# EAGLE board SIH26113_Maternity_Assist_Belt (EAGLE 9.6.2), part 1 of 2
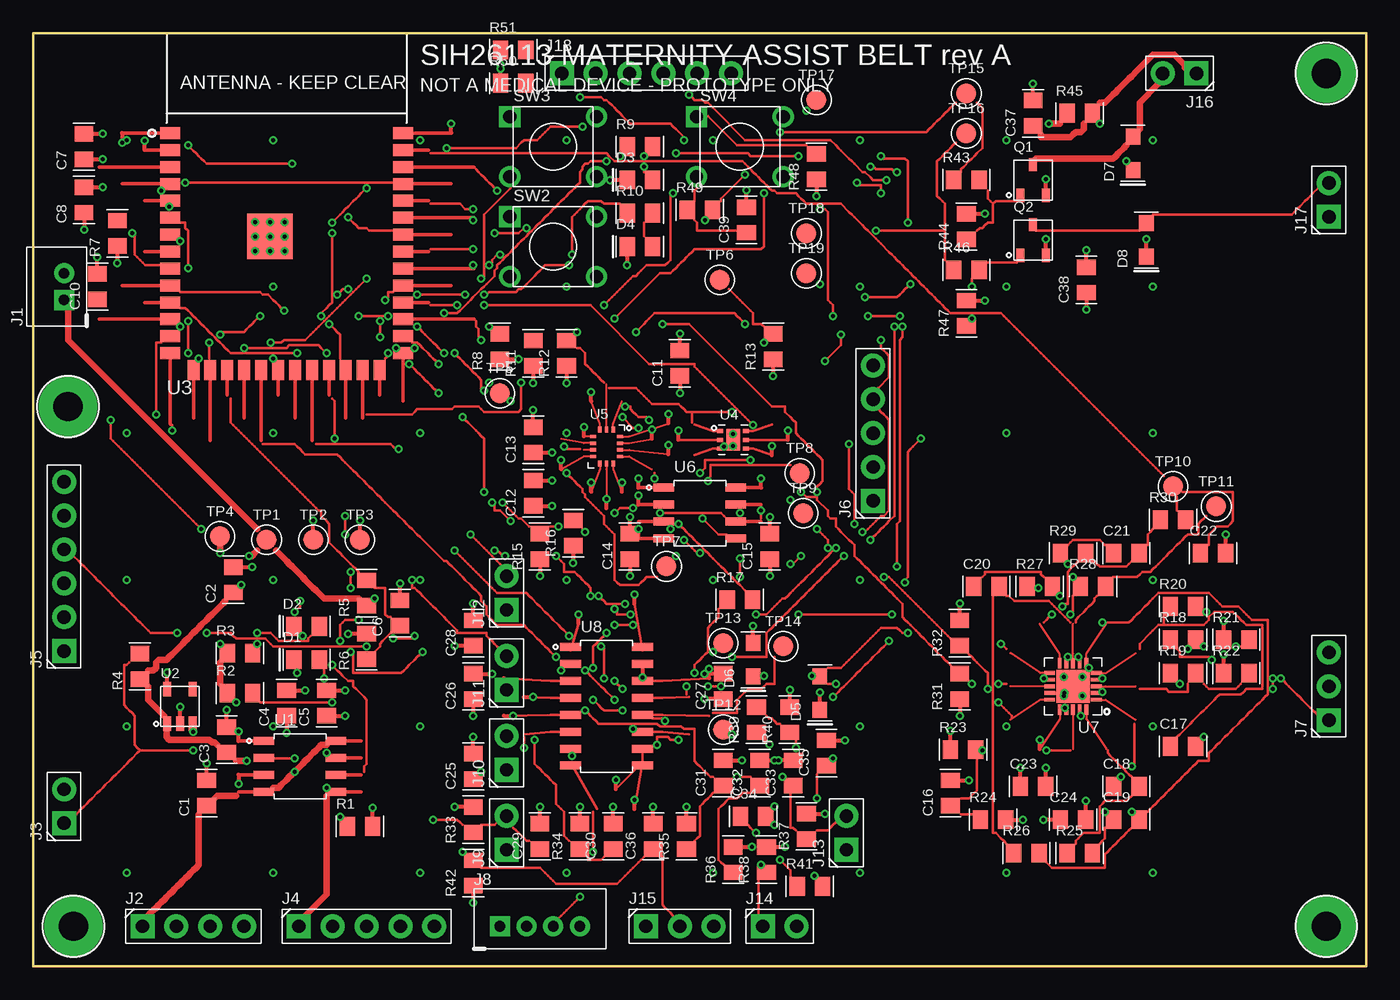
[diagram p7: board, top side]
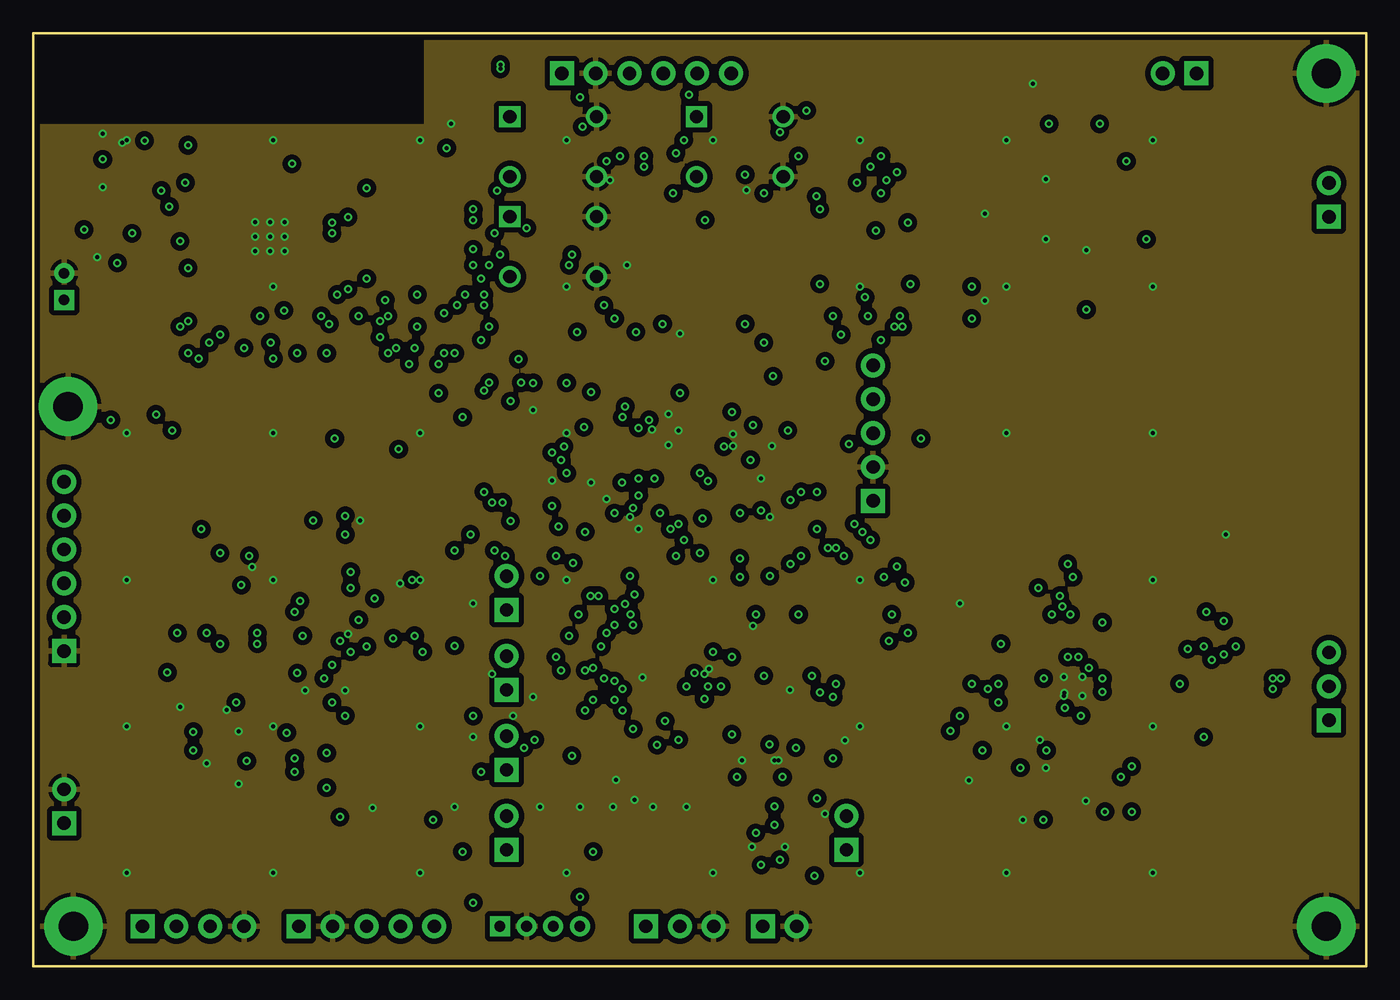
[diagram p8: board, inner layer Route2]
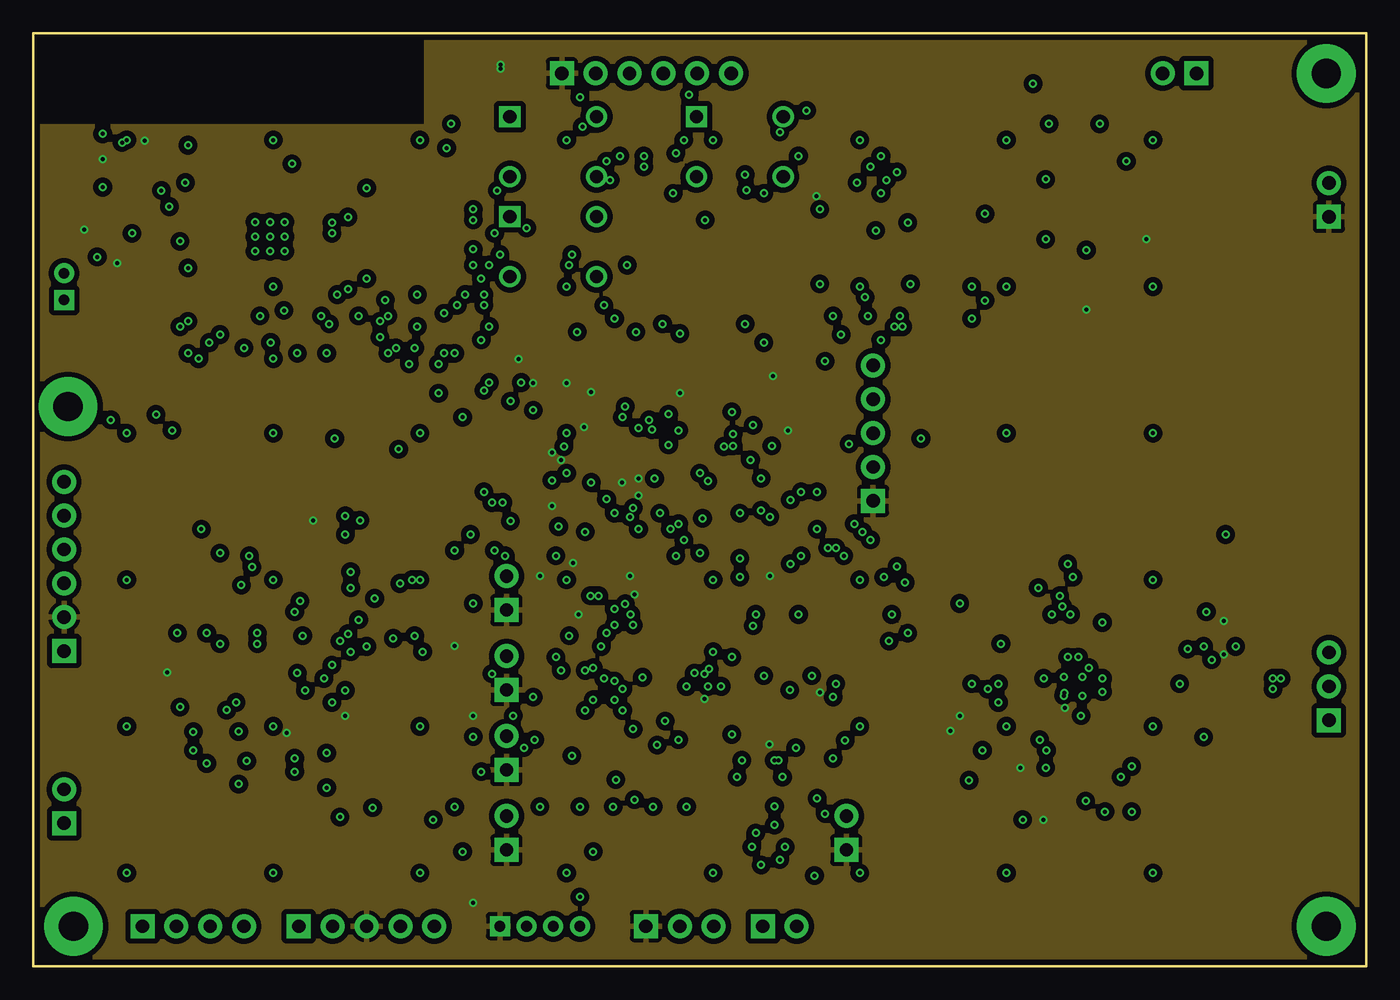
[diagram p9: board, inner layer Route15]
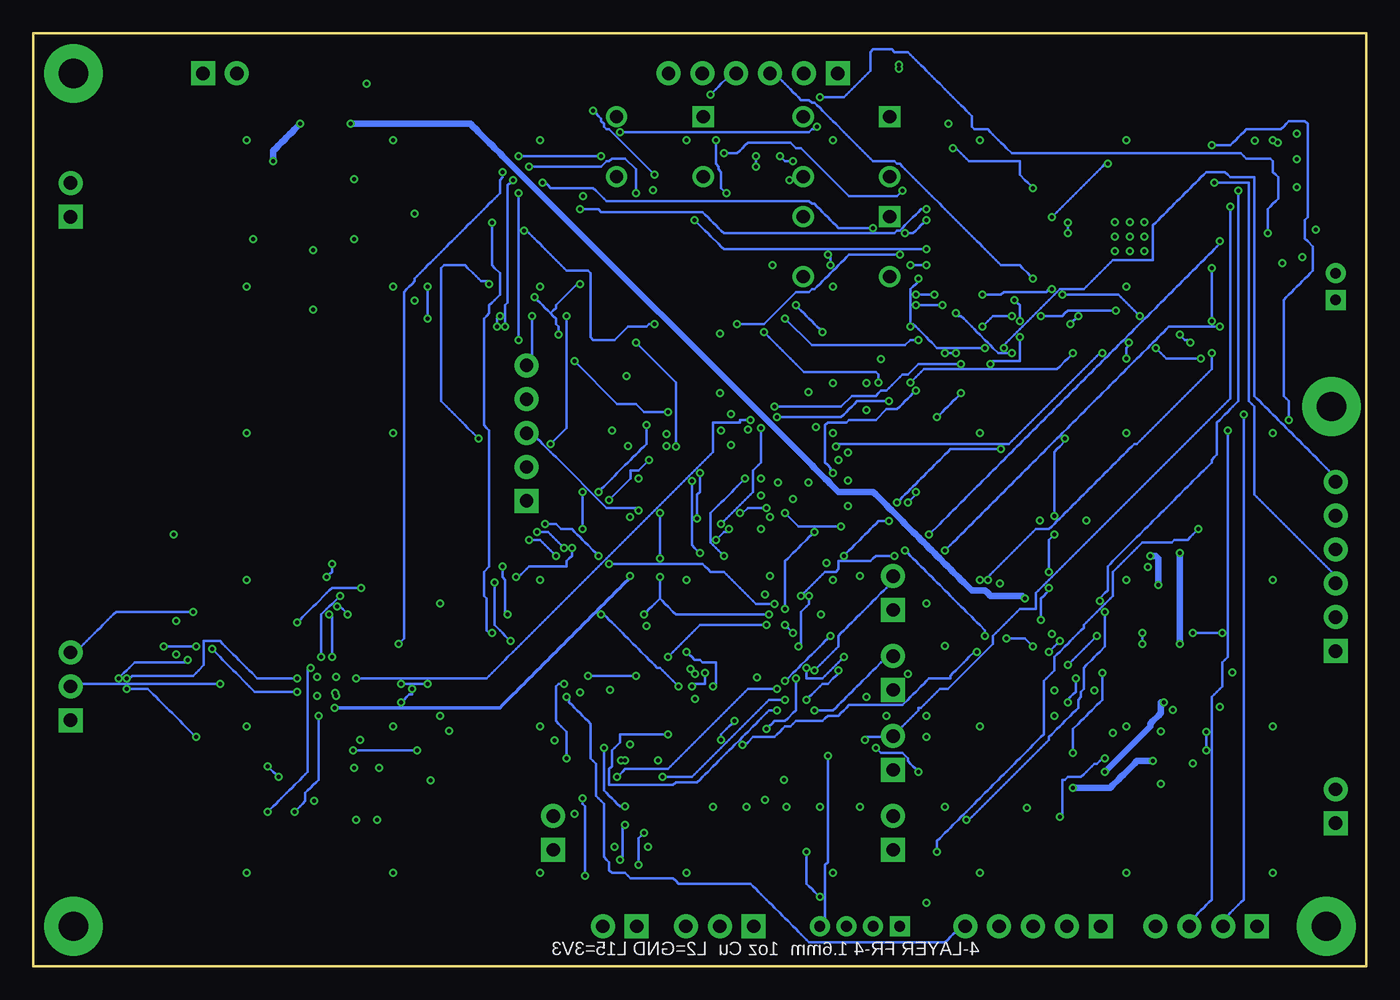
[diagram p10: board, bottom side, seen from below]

Size 100 x 70 mm. Coordinates in mm from the lower left corner, seen from the top.
Outline: 0,0 100,0 100,70 0,70 0,0
Copper layers (1*2*15*16): Top 0.035mm / dielectric 0.36mm / Route2 0.035mm / dielectric 0.71mm / Route15 / Bottom
Design rules "SIH26113_4layer": minimum track width 0.15mm, minimum drill 0.3mm, track to track 0.127mm, track to pad 0.127mm, pad to pad 0.127mm, via to via 0.127mm, smd to smd 0.127mm, copper to edge 0.4mm, drill to drill 0.25mm, minimum pad ring 0.25mm, minimum via ring 0.15mm, thermal gap 0.3mm
Net classes: 0 default: width 0.2 mm, drill 0.3 mm, clearance 0.15 mm; 1 power: width 0.5 mm, drill 0.4 mm, clearance 0.2 mm; 2 motor: width 0.5 mm, drill 0.4 mm, clearance 0.2 mm; 3 analog_ecg: width 0.2 mm, drill 0.3 mm, clearance 0.2 mm
tKeepout: 4 lines
bKeepout: 4 lines
tRestrict: 4 lines
bRestrict: 4 lines
vRestrict: 4 lines

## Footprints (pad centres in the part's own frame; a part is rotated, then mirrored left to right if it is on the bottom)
C0805 = smd 1.15 x 1.4: 1 -0.95,0; 2 0.95,0
LED0805 = smd 1.15 x 1.4: 1 -0.95,0; 2 0.95,0
SOD-123 = smd 1.2 x 1.1: 1 -1.25,0; 2 1.25,0
MOUNT-M2 = drill 2.2 pad 4.4: 1 0,0
JST-PH-2 = drill 0.8 pad 1.5 square: 1 -1,0 | drill 0.8 pad 1.5: 2 1,0
HDR-1X4 = drill 1 pad 1.8 square: 1 -3.81,0 | drill 1 pad 1.8: 2 -1.27,0; 3 1.27,0; 4 3.81,0
HDR-1X2 = drill 1 pad 1.8 square: 1 -1.27,0 | drill 1 pad 1.8: 2 1.27,0
HDR-1X5 = drill 1 pad 1.8 square: 1 -5.08,0 | drill 1 pad 1.8: 2 -2.54,0; 3 0,0; 4 2.54,0; 5 5.08,0
HDR-1X6 = drill 1 pad 1.8 square: 1 -6.35,0 | drill 1 pad 1.8: 2 -3.81,0; 3 -1.27,0; 4 1.27,0; 5 3.81,0; 6 6.35,0
HDR-1X3 = drill 1 pad 1.8 square: 1 -2.54,0 | drill 1 pad 1.8: 2 0,0; 3 2.54,0
JST-PH-4 = drill 0.8 pad 1.5 square: 1 -3,0 | drill 0.8 pad 1.5: 2 -1,0; 3 1,0; 4 3,0
SOT-23-3 = smd 0.6 x 1: 1 -0.95,-1.15; 2 0.95,-1.15; 3 0,1.15
R0805 = smd 1.15 x 1.4: 1 -0.95,0; 2 0.95,0
TACT-6X6-THT = drill 1 pad 1.6 square: 1 -3.25,2.25 | drill 1 pad 1.6: 2 -3.25,-2.25; 3 3.25,2.25; 4 3.25,-2.25
TESTPOINT-1.5 = smd 1.5 x 1.5: TP 0,0
SOIC-8-N = smd 1.55 x 0.6: 1 -2.7,1.905; 2 -2.7,0.635; 3 -2.7,-0.635; 4 -2.7,-1.905; 5 2.7,-1.905; 6 2.7,-0.635; 7 2.7,0.635; 8 2.7,1.905
SOT-23-5 = smd 0.6 x 1.1: 1 -0.95,-1.3; 2 0,-1.3; 3 0.95,-1.3; 4 0.95,1.3; 5 -0.95,1.3
ESP32-S3-WROOM-1 = smd 1.5 x 0.9: 1 -8.75,5.26; 2 -8.75,3.99; 3 -8.75,2.72; 4 -8.75,1.45; 5 -8.75,0.18; 6 -8.75,-1.09; 7 -8.75,-2.36; 8 -8.75,-3.63; 9 -8.75,-4.9; 10 -8.75,-6.17; 11 -8.75,-7.44; 12 -8.75,-8.71; 13 -8.75,-9.98; 14 -8.75,-11.25; 27 8.75,-11.25; 28 8.75,-9.98; 29 8.75,-8.71; 30 8.75,-7.44; 31 8.75,-6.17; 32 8.75,-4.9; 33 8.75,-3.63; 34 8.75,-2.36; 35 8.75,-1.09; 36 8.75,0.18; 37 8.75,1.45; 38 8.75,2.72; 39 8.75,3.99; 40 8.75,5.26 | smd 0.9 x 1.5: 15 -6.985,-12.5; 16 -5.715,-12.5; 17 -4.445,-12.5; 18 -3.175,-12.5; 19 -1.905,-12.5; 20 -0.635,-12.5; 21 0.635,-12.5; 22 1.905,-12.5; 23 3.175,-12.5; 24 4.445,-12.5; 25 5.715,-12.5; 26 6.985,-12.5 | smd 3.4 x 3.4: 41 -1.25,-2.5
WSON-6-DRV0006B = smd 0.45 x 0.3: 1 -0.975,0.65; 2 -0.975,0; 3 -0.975,-0.65; 4 0.975,-0.65; 5 0.975,0; 6 0.975,0.65 | smd 1 x 1.6: 7 0,0
LGA-14L-2.5X3.0 = smd 0.45 x 0.25: 1 1.025,0.75; 2 1.025,0.25; 3 1.025,-0.25; 4 1.025,-0.75; 8 -1.025,-0.75; 9 -1.025,-0.25; 10 -1.025,0.25; 11 -1.025,0.75 | smd 0.25 x 0.45: 5 0.5,-1.275; 6 0,-1.275; 7 -0.5,-1.275; 12 -0.5,1.275; 13 0,1.275; 14 0.5,1.275
LFCSP-20-4X4-P050 = smd 0.8 x 0.28: 1 -1.75,1; 2 -1.75,0.5; 3 -1.75,0; 4 -1.75,-0.5; 5 -1.75,-1; 11 1.75,-1; 12 1.75,-0.5; 13 1.75,0; 14 1.75,0.5; 15 1.75,1 | smd 0.28 x 0.8: 6 -1,-1.75; 7 -0.5,-1.75; 8 0,-1.75; 9 0.5,-1.75; 10 1,-1.75; 16 1,1.75; 17 0.5,1.75; 18 0,1.75; 19 -0.5,1.75; 20 -1,1.75 | smd 2.5 x 2.5: EP 0,0
SOP-16-N = smd 1.55 x 0.6: 1 -2.7,4.445; 2 -2.7,3.175; 3 -2.7,1.905; 4 -2.7,0.635; 5 -2.7,-0.635; 6 -2.7,-1.905; 7 -2.7,-3.175; 8 -2.7,-4.445; 9 2.7,-4.445; 10 2.7,-3.175; 11 2.7,-1.905; 12 2.7,-0.635; 13 2.7,0.635; 14 2.7,1.905; 15 2.7,3.175; 16 2.7,4.445

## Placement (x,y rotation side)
C1  10u  [C0805]  13,13 90 top
C2  10u  [C0805]  15,29 90 top
C3  10u  [C0805]  14.5,17 90 top
C4  10u  [C0805]  19,19.75 90 top
C5  100n  [C0805]  22,19.75 90 top
C6  100n  [C0805]  27.5,26.5 90 top
C7  100n  [C0805]  3.8,61.5 90 top
C8  22u  [C0805]  3.8,57.5 90 top
C10  1u  [C0805]  4.8,51 90 top
C11  100n  [C0805]  48.5,45.25 90 top
C12  100n  [C0805]  37.5,35.5 90 top
C13  100n  [C0805]  37.5,39.5 90 top
C14  100n  [C0805]  44.75,31.5 90 top
C15  1u  [C0805]  55.25,31.5 90 top
C16  100n  [C0805]  68.8,13 90 top
C17  1n  [C0805]  86.25,16.5 0 top
C18  220n  [C0805]  82,13.5 0 top
C19  220n  [C0805]  82,11 0 top
C20  8n2  [C0805]  71.5,28.5 0 top
C21  3n9  [C0805]  82,31 0 top
C22  10n  [C0805]  88.5,31 0 top
C23  100n  [C0805]  75,13.5 0 top
C24  1u  [C0805]  78,11 0 top
C25  100n  [C0805]  33,15 90 top
C26  100n  [C0805]  33,21 90 top
C27  100n  [C0805]  51.75,21 90 top
C28  10u  [C0805]  33,25 90 top
C29  10n  [C0805]  38,9.75 90 top
C30  10n  [C0805]  43.5,9.75 90 top
C31  10n  [C0805]  51.75,14.5 90 top
C32  10n  [C0805]  54.5,14.5 90 top
C33  10n  [C0805]  57,14.5 90 top
C34  100n/50V  [C0805]  54,11.25 0 top
C35  10n  [C0805]  59.5,16 90 top
C36  100n  [C0805]  46.5,9.75 90 top
C37  10u  [C0805]  75,64 90 top
C38  10u  [C0805]  79,51.5 90 top
C39  100n  [C0805]  53.5,56 90 top
D1  RED  [LED0805]  20.5,23 0 top
D2  GRN  [LED0805]  20.5,25.5 0 top
D3  GRN  [LED0805]  45.5,59 0 top
D4  RED  [LED0805]  45.5,54 0 top
D5  1N5819HW  [SOD-123]  59,20.5 90 top
D6  1N5819HW  [SOD-123]  54,23 90 top
D7  1N5819HW  [SOD-123]  82.5,61 90 top
D8  1N5819HW  [SOD-123]  83.5,54.5 90 top
H1  M2  [MOUNT-M2]  3,3 0 top
H2  M2  [MOUNT-M2]  97,3 0 top
H3  M2  [MOUNT-M2]  2.6,42 0 top
H4  M2  [MOUNT-M2]  97,67 0 top
J1  LI-PO 3.7V  [JST-PH-2]  2.3,51 90 top
J2  USB / 5V IN  [HDR-1X4]  12,3 0 top
J3  OFF SW  [HDR-1X2]  2.3,12 90 top
J4  FUEL GAUGE  [HDR-1X5]  25,3 0 top
J5  UART PROG  [HDR-1X6]  2.3,30 90 top
J6  AS5600 SIDE-B  [HDR-1X5]  63,40 90 top
J7  ECG ELECTRODES  [HDR-1X3]  97.2,21 90 top
J8  LOAD CELL  [JST-PH-4]  38,3 0 top
J9  FSR1  [HDR-1X2]  35.5,10 90 top
J10  FSR2  [HDR-1X2]  35.5,16 90 top
J11  FSR3  [HDR-1X2]  35.5,22 90 top
J12  FSR4  [HDR-1X2]  35.5,28 90 top
J13  STRETCH  [HDR-1X2]  61,10 90 top
J14  PIEZO  [HDR-1X2]  56,3 0 top
J15  HALL / LIMIT  [HDR-1X3]  48.5,3 0 top
J16  VIB MOTOR  [HDR-1X2]  86,67 180 top
J17  BUZZER  [HDR-1X2]  97.2,57.5 90 top
J18  MICROSD SPI  [HDR-1X6]  46,67 0 top
Q1  AO3400A  [SOT-23-3]  75,59 0 top
Q2  AO3400A  [SOT-23-3]  75,54.5 0 top
R1  2k4  [R0805]  24.5,10.5 0 top
R2  1k  [R0805]  15.5,20.5 0 top
R3  1k  [R0805]  15.5,23.5 0 top
R4  100k  [R0805]  8,22.5 90 top
R5  470k  [R0805]  25,28 90 top
R6  470k  [R0805]  25,24 90 top
R7  10k  [R0805]  6.3,55 90 top
R8  10k  [R0805]  35,46.5 90 top
R9  1k  [R0805]  45.5,61.5 0 top
R10  1k  [R0805]  45.5,56.5 0 top
R11  4k7  [R0805]  37.5,46 90 top
R12  4k7  [R0805]  40,46 90 top
R13  10k  [R0805]  55.5,46.5 90 top
R15  4k7  [R0805]  38,31.5 90 top
R16  4k7  [R0805]  40.5,32.5 90 top
R17  0R DNP  [R0805]  53,27.5 0 top
R18  330k  [R0805]  86.25,24.5 0 top
R19  330k  [R0805]  86.25,22 0 top
R20  330k  [R0805]  86.25,27 0 top
R21  10M  [R0805]  90.25,24.5 0 top
R22  10M  [R0805]  90.25,22 0 top
R23  10M  [R0805]  69.75,16.25 0 top
R24  10M  [R0805]  72,11 0 top
R25  10M  [R0805]  78.5,8.5 0 top
R26  1M  [R0805]  74.5,8.5 0 top
R27  470k  [R0805]  75.5,28.5 0 top
R28  100k  [R0805]  79.5,28.5 0 top
R29  1M  [R0805]  78,31 0 top
R30  1k  [R0805]  85.5,33.5 0 top
R31  100k  [R0805]  69.5,21 90 top
R32  100k  [R0805]  69.5,25 90 top
R33  10k  [R0805]  33,11 90 top
R34  10k  [R0805]  41,9.75 90 top
R35  10k  [R0805]  49,9.75 90 top
R36  10k  [R0805]  52.5,8 90 top
R37  10k  [R0805]  58,10.5 90 top
R38  10M  [R0805]  55,8 90 top
R39  1M  [R0805]  54.25,18.5 90 top
R40  1M  [R0805]  56.75,18.5 90 top
R41  100k  [R0805]  58.25,6 0 top
R42  10k  [R0805]  33,7 90 top
R43  100R  [R0805]  70,59 0 top
R44  100k  [R0805]  70,55.5 90 top
R45  0R  [R0805]  78.5,64 0 top
R46  100R  [R0805]  70,52.25 0 top
R47  100k  [R0805]  70,49 90 top
R48  10k  [R0805]  58.75,60 90 top
R49  1k  [R0805]  50,56.75 0 top
R50  10k  [R0805]  36,66.25 0 top
R51  10k  [R0805]  36,68.75 0 top
SW2  RESET  [TACT-6X6-THT]  39,54 0 top
SW3  BOOT  [TACT-6X6-THT]  39,61.5 0 top
SW4  SOS  [TACT-6X6-THT]  53,61.5 0 top
TP1  VBAT  [TESTPOINT-1.5]  17.5,32 0 top
TP2  3V3  [TESTPOINT-1.5]  21,32 0 top
TP3  GND  [TESTPOINT-1.5]  24.5,32 0 top
TP4  VBUS  [TESTPOINT-1.5]  14,32.25 0 top
TP5  IO3  [TESTPOINT-1.5]  35,43 0 top
TP6  TMP_ALERT  [TESTPOINT-1.5]  51.5,51.5 0 top
TP7  IMU_INT1  [TESTPOINT-1.5]  47.5,30 0 top
TP8  AS_OUT  [TESTPOINT-1.5]  57.5,37 0 top
TP9  AS_PGO  [TESTPOINT-1.5]  57.75,34 0 top
TP10  ECG_OUT  [TESTPOINT-1.5]  85.5,36 0 top
TP11  ECG_REF  [TESTPOINT-1.5]  88.75,34.5 0 top
TP12  HX_BASE  [TESTPOINT-1.5]  51.75,17.75 0 top
TP13  HX_XO  [TESTPOINT-1.5]  51.75,24.25 0 top
TP14  HX_DOUT  [TESTPOINT-1.5]  56.25,24 0 top
TP15  MOTOR_EN  [TESTPOINT-1.5]  70,65.5 0 top
TP16  BUZZER_EN  [TESTPOINT-1.5]  70,62.5 0 top
TP17  SOS_GPIO  [TESTPOINT-1.5]  58.75,65 0 top
TP18  I2C_SDA  [TESTPOINT-1.5]  58,55 0 top
TP19  I2C_SCL  [TESTPOINT-1.5]  58,52 0 top
U1  TP4056  [SOIC-8-N]  20,15 0 top
U2  AP2112K-3.3  [SOT-23-5]  11,19.5 0 top
U3  ESP32-S3-WROOM-1-N8R2  [ESP32-S3-WROOM-1]  19,57.25 0 top
U4  TMP117  [WSON-6-DRV0006B]  52.5,39.5 0 top
U5  LSM6DSOX  [LGA-14L-2.5X3.0]  43,39 0 top
U6  AS5600  [SOIC-8-N]  50,34 0 top
U7  AD8232  [LFCSP-20-4X4-P050]  78,21 180 top
U8  HX711  [SOP-16-N]  43,19.5 0 top

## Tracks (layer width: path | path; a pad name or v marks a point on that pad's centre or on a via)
3V3  (via drill 0.3 pad 0.55, 0.3 pad 0.6)
  Top 0.15: U5.5 43.5,37.3 44.15,35.6 | U5.8 41.3,38.25 39.6,37.27 | U5.11 41.3,39.75 | U5.12 42.5,40.7 41.85,42.4
  Top 0.2: U4.5 54,39.5 56.6,39.5 | U8.1 40.3,23.7 40.9,25.7 | U8.16 45.7,23.7 45.1,27.2 | U8.3 38.8,21.41 35.3,21.6
  Top 0.25: U3.2 8.35,61.24 | U6.1 45.4,35.91 | U6.2 45.4,34.63
  Top 0.3: U2.5 v10.05,22.05 | C4.1 v19,17.52 | C5.1 v23.4,18.8 | TP2.TP v21,33.45 | 8.35,61.24 v8.35,61.94 | C7.1 v5.2,60.55 | C8.1 v3.8,55.27 | R7.1 v6.3,52.77 | R8.1 v36.4,45.55 | R11.1 v37.5,43.77 | R12.1 v40,43.77 | 56.6,39.5 v56.6,40.2 | C11.1 v48.5,43.02 | R13.1 v55.5,44.27 | 44.15,35.6 v44.15,36.3 | 39.6,37.27 v39.6,37.98 | 41.3,39.75 v41.3,40.45 | 41.85,42.4 v41.85,43.1 | C12.1 v38.9,34.55 | C13.1 v38.9,38.55 | R15.1 v38,29.27 | R16.1 v40.5,30.27 | 45.4,35.91 v45.4,36.6 | 45.4,34.63 v45.4,35.34 | C14.1 v44.75,29.27 | C15.1 v55.25,29.27 | R21.1 v89.3,25.9 | R22.1 v89.3,23.4 | R23.1 v68.8,17.65 | R31.1 v69.5,18.77 | C23.1 v74.05,14.9 | C24.1 v75.78,11 | 40.9,25.7 v40.9,26.4 | 35.3,21.6 v35.3,20.9 | 45.1,27.2 v45.1,27.9 | C26.1 v33,18.77 | C27.1 v50.35,20.05 | C28.1 v31.6,24.05 | R39.1 v55.24,16.64 | D5.1 v59,20.55 | R42.1 v33,4.78 | D8.1 v83.5,54.55 | C38.1 v79,49.27 | R48.1 v58.75,57.77 | R50.1 v35.05,67.65 | R51.1 v35.05,67.35
  Bottom 0.25: v77.4,19.4 65,19.4 64.8,19.6 64.6,19.8 64.4,20 64.2,20.2 64,20.4 63.8,20.6 63.6,20.8 63.4,21 63.2,21.2 63,21.4 62.8,21.6 62.6,21.8 62.4,22 62.2,22.2 62,22.4 61.8,22.6 61.6,22.8 61.4,23 61.2,23.2 61,23.4 60.8,23.6 60.6,23.8 60.4,24 60.2,24.2 60,24.4 59.8,24.6 59.6,24.8 59.4,25 59.2,25.2 59,25.4 58.8,25.6 58.6,25.8 58.4,26 58.2,26.2 58,26.4 57.8,26.6 57.6,26.8 57.4,27 57.2,27.2 57,27.4 56.8,27.6 56.6,27.8 56.4,28 56.2,28.2 56,28.4 55.8,28.6 55.6,28.8 55.4,29
  pour Route15 (isolate 0.4): 0.5,0.5 99.5,0.5 99.5,69.5 29.5,69.5 29.5,63 0.5,63
ANG2_OUT  (via drill 0.3 pad 0.6)
  Top 0.2: 51.4,26.8 51.4,26.2 51.2,26 51,25.8 50.8,25.6 50.6,25.4 50.6,23.6 50.4,23.4 50.2,23.2 50,23 49.8,22.8 49.6,22.6 v49.6,22 | v50.6,21 v51.6,21 | v57.4,26.4 v64.4,26.4 | v64.8,30 64.8,33.2 65,33.4 65,47 65.2,47.2 v65.2,48 | v65,48.8 v62.6,48.8
  Bottom 0.2: v49.6,22 49.6,21.2 50.4,21.2 v50.6,21 | v51.6,21 51.8,21.2 52,21.4 52.4,21.8 52.6,22 52.8,22.2 53,22.4 53.2,22.4 53.4,22.6 53.6,22.8 53.8,23 54,23.2 54.4,23.6 54.6,23.8 54.8,24 55,24.2 55.4,24.6 55.6,24.8 55.8,25 56,25.2 56.4,25.6 56.6,25.8 56.8,26 57,26.2 57.2,26.4 v57.4,26.4 | v64.4,26.4 64.6,26.6 64.6,29 64.8,29.2 v64.8,30 | v65.2,48 65.2,48.6 v65,48.8 | v62.6,48.8 62.6,45.8
ANG_SCL  (via drill 0.3 pad 0.6)
  Top 0.2: 53,34.4 v53,34 | v53,30.6 v53,29.2 | v54.2,26.4 55,26.4 55.4,26.8 55.6,27 55.8,27.2 56,27.4 56.2,27.6 56.4,27.6 56.6,27.8 56.8,28 57,28.2 57.4,28.6 57.6,28.8 57.8,29 58,29.2 58.4,29.6 58.6,29.8 58.8,30 59,30.2 59.4,30.6 59.6,30.8 59.8,31 60,31.2 v60.2,31.4 | v62.2,32.6 62.4,32.6 62.6,32.8 62.8,33 63,33.2 63.2,33.4 63.4,33.6 63.6,33.8 63.8,33.8 64.2,34.2 64.2,41 64,41.2 63.8,41.4 63.6,41.6 63.4,41.8 | 41.2,32.8 v41.4,32.6 | v43.6,26.8 43.8,26.6 43.8,26.4 v44.8,26.4 | v34.6,55 36.4,55 36.8,55.4 v37,55.4 | v61.8,58.8 62,58.6 63.6,58.6 v63.6,58 | v63.6,47 63.6,46.4 63.8,46.2 64,46 64.2,45.8 64.2,44.2 63.4,43.4
  Top 0.25: U3.35 33.05,56.16 | U6.7 54.6,34.63
  Bottom 0.2: v53,34 v53,30.6 | v53,29.2 53,27.6 | 53,27.6 53.4,27.2 53.6,27 53.8,26.8 54,26.6 v54.2,26.4 | v60.2,31.4 60.4,31.6 60.6,31.8 60.8,32 61,32.2 61.2,32.4 61.4,32.6 v62.2,32.6 | v41.4,32.6 41.6,32.4 41.8,32.2 42,32 42.4,31.6 42.6,31.4 42.8,31.2 43,31 43.4,30.6 43.6,30.4 v43.6,26.8 | v44.8,26.4 51.8,26.4 52,26.6 52.4,27 52.6,27.2 52.8,27.4 53,27.6 | v33,56 33.2,55.8 33.4,55.6 33.6,55.4 33.8,55.2 34,55 v34.6,55 | v37,55.4 39.6,55.4 39.8,55.6 40,55.8 40.2,56 40.4,56.2 40.6,56.4 40.8,56.6 41,56.8 41.2,57 41.4,57.2 41.6,57.2 41.8,57.4 57,57.4 57.2,57.6 57.8,58.2 58,58.4 61.2,58.4 61.4,58.6 61.6,58.8 v61.8,58.8 | v63.6,58 v63.6,47
ANG_SDA  (via drill 0.3 pad 0.6)
  Top 0.2: 54.6,33.6 v54.6,34.2 | 38.8,33 v39.4,33 | v43.6,34 44,34.4 v45,34.4 | v47,34 51.6,34 51.8,33.8 52,33.6 | 21.2,39.2 26.8,39.2 27,39 27.2,38.8 v27.4,38.8 | v35.2,34.8 35.4,34.6 35.6,34.4 35.8,34.2 36,34 36.2,33.8 36.4,33.6 36.6,33.6 37.2,33
  Top 0.25: U3.22 20.91,39.45 | U6.6 54.6,33.37
  Bottom 0.2: v54.6,34.2 54.6,34.4 57,34.4 60.8,38.2 61,38.4 61.2,38.6 61.8,39.2 62,39.4 62.2,39.6 | v39.4,33 42.6,33 v43.6,34 | v45,34.4 46.4,34.4 46.8,34 v47,34 | v27.4,38.8 31.2,38.8 31.4,38.6 31.6,38.4 32,38 32.2,37.8 32.4,37.6 32.6,37.4 32.8,37.2 33,37 33.2,36.8 33.4,36.6 33.6,36.4 33.8,36.2 34,36 34.2,35.8 34.4,35.6 34.6,35.4 34.8,35.2 35,35 v35.2,34.8
AS_OUT  (via drill 0.3 pad 0.6)
  Top 0.2: 47.8,33 v47.8,32.8 | v48.8,32 49,31.8 49.4,31.4 49.6,31.2 49.8,31 v50,31 | v50.6,36.4 50.6,36.6 50.8,36.8 50.8,37.6 56.8,37.6
  Top 0.25: U6.3 45.4,33.37
  Bottom 0.2: v47.8,32.8 47.8,32.6 48.2,32.6 v48.8,32 | v50,31 50.2,31.2 50.4,31.4 50.6,31.6 v50.6,36.4
AS_PGO  (via drill 0.3 pad 0.6)
  Top 0.2: 52,32.4 51.4,32.4 v50.2,33.6 | v50,37 50.2,37.2 50.4,37.4 50.4,38 v53.8,38 | v56.8,35 57,34.8
  Bottom 0.2: v50.2,33.6 50.2,35.4 50,35.6 v50,37 | v53.8,38 54.6,37.2 55.2,37.2 55.2,36.6 v56.8,35
BUZZ_G  (via drill 0.3 pad 0.6)
  Top 0.2: 70.4,51.6 v70.4,51 | 73.8,52.8 71.6,52.8
  Bottom 0.2: v70.4,51 v70.4,48.6
BUZZ_N
  Top 0.2: 84,56.4 94.4,56.4 94.6,56.6 94.8,56.8 95,57 95.4,57.4 95.6,57.6 95.8,57.8 96,58 96.4,58.4 | 75.2,55.2 83,55.2
BUZZER_EN  (via drill 0.3 pad 0.6)
  Top 0.2: 68.4,53 68.4,57.2 68.2,57.4 68,57.6 67.8,57.8 67.8,60.4 68,60.6 68.2,60.8 68.4,61 68.6,61.2 68.8,61.4 69,61.6 69.2,61.8 | 25,41.4 28.4,41.4 28.6,41.6 28.8,41.8 31.4,41.8 31.6,42 33.4,42 33.6,41.8 33.8,41.6 36.4,41.6 36.6,41.8 v36.6,43.8 | v45.2,47.6 45.8,48.2 46,48.4 46.2,48.6 46.6,49 52.6,49 52.8,48.8 53,48.6 53.2,48.4 v53.4,48.2 | v63.2,55.2 68.4,55.2
  Top 0.25: U3.25 24.71,41.15
  Bottom 0.2: v36.6,43.8 36.6,44.4 36.8,44.6 42.2,44.6 42.8,45.2 43,45.4 43.2,45.6 43.8,46.2 44,46.4 44.2,46.6 44.8,47.2 45,47.4 v45.2,47.6 | v53.4,48.2 53.8,48.2 54,48 55.4,48 56.4,47 58,47 58.2,47.2 58.2,52 58.4,52.2 60,52.2 60.2,52.4 60.4,52.6 60.6,52.8 60.8,53 61,53.2 61.2,53.4 61.4,53.6 61.6,53.8 61.8,54 62,54.2 62.2,54.4 62.4,54.6 62.6,54.8 62.8,55 63,55.2 v63.2,55.2
CHG_PROG  (via drill 0.3 pad 0.6)
  Top 0.2: 18,15.6 v19.6,15.6
  Bottom 0.2: v19.6,15.6 19.8,15.6 20,15.4 20.2,15.2 20.4,15.2 20.6,15 21,14.6 21.2,14.4 21.4,14.2 22.4,14.2 22.6,14 22.8,14 22.8,11.4 v23,11.2
ECG_FR  (via drill 0.3 pad 0.6)
  Top 0.15: U7.15 75.55,20 73.3,18.5
  Top 0.2: 73.4,18.6 73.4,18.8 73.2,19 73,19.2 72.8,19.4 72.6,19.6 v72.4,19.8 | v71.6,20.8 71.6,22 71.4,22.2 70.8,22.8 70.6,23 70.4,23.2 70.2,23.4 | v34.2,52.6 34.4,52.8 34.4,53 34.8,53.4 v35,53.4 | v47.2,48.2 49.2,48.2 55.4,42 56.4,42 56.4,41.6 56.8,41.2 57,41 57.2,40.8 57.2,40 57.4,39.8 57.6,39.6 57.8,39.4 58,39.2 58.2,39 58.4,38.8 58.6,38.6 58.8,38.4 59,38.2 59.2,38 59.2,36.4 59,36.2 58.8,36 v58.8,35.6 | v58.8,32.8 59,32.6 59.2,32.4 59.4,32.2 59.6,32 v59.6,31.4 | v63.8,29.2 64.2,29.2 64.4,29 64.6,28.8 64.8,28.6 65.2,28.2 65.4,28 65.6,27.8 65.8,27.6 66.2,27.2 66.4,27 66.6,26.8 66.8,26.6 67.2,26.2 67.4,26 67.6,25.8 67.8,25.6 68.2,25.2 68.4,25 68.6,24.8 68.8,24.6
  Top 0.25: U3.32 33.05,52.35
  Bottom 0.2: v72.4,19.8 72.2,20 72,20.2 71.8,20.4 71.6,20.4 v71.6,20.8 | v33,52.6 v34.2,52.6 | v35,53.4 38.8,53.4 39,53.2 39.2,53 39.4,52.8 39.6,52.6 39.8,52.4 40,52.2 40.2,52 40.4,51.8 40.6,51.6 40.8,51.4 41,51.2 41.2,51 41.4,50.8 41.6,50.8 41.8,50.6 42.8,50.6 45.2,48.2 v47.2,48.2 | v58.8,35.6 v58.8,32.8 | v59.6,31.4 59.6,30.8 59.8,30.6 60,30.4 60,30 62.8,30 63,29.8 63.4,29.4 63.6,29.2 v63.8,29.2
ECG_HPDRIVE  (via drill 0.3 pad 0.6)
  Top 0.15: U7.1 80.45,20 82.7,18.5
  Top 0.2: 82.6,18.2 82.6,15.2 v82.4,15
  Bottom 0.2: v82.4,15 82,14.6 81.8,14.4 v81.6,14.2
ECG_HPSENSE
  Top 0.15: U7.20 79,18.55 80.5,16.3
  Top 0.2: 80.6,16.2 80.6,16 80.8,15.8 81,15.6 81.2,15.4 81.4,15.2 81.6,15 81.8,14.8 82,14.6 82.2,14.4 82.4,14.2 | 78.2,9.2 78.2,9.4 78.4,9.6 78.8,10 80,10 80,12 80.2,12.2 80.4,12.4 82,12.4 82.2,12.6 82.4,12.8
ECG_IAOUT  (via drill 0.3 pad 0.6)
  Top 0.2: 80.4,9.6 80.4,10.4 80.4,9.6 | 80.4,9.6 80.2,9.4 | 80.2,9.4 80,9.2 80.2,9.4 | 80.4,9.6 80.2,9.4
  Bottom 0.2: v78.6,18.8 78.6,14 78.8,13.8 79,13.6 79.2,13.4 79.4,13.2 79.6,13 79.6,12.4 79.8,12.2 80,12 v80.4,11.6
ECG_LA  (via drill 0.3 pad 0.6)
  Top 0.2: 85.8,23.8 86,23.6 86,23.2 88.2,23.2 v88.4,23 | v93.6,21.6 93.8,21.4 94,21.2 94.2,21 94.8,20.4 95,20.2 95.2,20 95.8,19.4 96,19.2 96.2,19 96.4,18.8
  Bottom 0.2: v88.4,23 88.6,22.8 92.4,22.8 92.8,22.4 93,22.2 93.2,22 v93.6,21.6
ECG_LA_F  (via drill 0.3 pad 0.6)
  Top 0.2: 90.6,24 v90.2,24
  Bottom 0.2: v90.2,24 v87.8,24 | v80.2,20.6 83.4,20.6 83.8,21 84,21.2 84.8,22 85,22.2 85.8,23 86,23.2 v86.6,23.8
ECG_LOD_N  (via drill 0.3 pad 0.6)
  Top 0.15: U7.11 75.55,22 73.3,23.5
  Top 0.2: 73,23.8 72.8,24 v72.6,24.2 | v64.8,59.6 64.6,59.6 64.4,59.8 63.2,59.8 63,60 v62.8,60 | v54.8,58 54.8,54 54.6,53.8 49.6,53.8 49.4,53.6 49.2,53.4 49,53.2 48.8,53 48.6,52.8 48.4,52.6 48.2,52.4 48,52.2 47.8,52 47,52 v43.6,48.6 | v33.6,47 33.4,47.2 33.4,47.8 33.2,48 33.2,48.4
  Top 0.25: U3.29 33.05,48.54
  Bottom 0.2: v72.6,24.2 72.2,24.6 72.2,50.6 72,50.8 71.8,51 71.6,51.2 71.4,51.4 71.4,51.6 71.2,51.8 71,52 70.8,52.2 70.6,52.4 70.4,52.6 70.2,52.8 70,53 69.8,53.2 69.6,53.4 69.4,53.6 69.2,53.8 69,54 68.8,54.2 68.6,54.4 68.4,54.6 68.2,54.8 68,55 67.8,55.2 67.6,55.4 67.4,55.6 67.2,55.8 67,56 66.8,56.2 66.6,56.4 66.4,56.6 66.2,56.8 66,57 65.8,57.2 65.6,57.4 65.4,57.6 65.2,57.8 65,58 65,59 64.8,59.2 v64.8,59.6 | v62.8,60 57.4,60 57,60.4 56.8,60.4 56.6,60.6 55.6,60.6 54.8,59.8 v54.8,58 | v43.6,48.6 41.6,46.6 34.6,46.6 34.2,47 v33.6,47
ECG_LOD_P  (via drill 0.3 pad 0.6)
  Top 0.2: v46.2,41 46,41.2 45.4,41.2 45.2,41.4 45,41.6 44.8,41.8 44.8,42 v44.4,42 | v30.4,45.2 30.2,45.4 30,45.6 29.8,45.8 29.6,46 29.2,46.4 29,46.6 28.8,46.8 28.4,46.8
  Bottom 0.2: v75.8,21.6 66,21.6 65.8,21.8 65.6,22 65.4,22.2 64.8,22.8 64.6,23 64.4,23.2 64,23.6 63.8,23.8 63.6,24 63.4,24.2 63,24.6 62.8,24.8 62.6,25 62.4,25.2 62,25.6 61.8,25.8 61.6,26 61.4,26.2 61,26.6 60.8,26.8 60.6,27 60.4,27.2 60,27.6 59.8,27.8 59.6,28 59.4,28.2 59,28.6 58.8,28.8 58.6,29 58.4,29.2 58,29.6 57.8,29.8 57.6,30 57.4,30.2 57,30.6 56.8,30.8 56.6,31 56.4,31.2 56,31.6 55.8,31.8 55.6,32 55.4,32.2 55.2,32.4 55,32.6 54.8,32.8 54.6,33 54.4,33.2 54.2,33.4 54,33.6 53.8,33.8 53.6,34 53.4,34.2 53.2,34.4 53,34.6 52.8,34.8 52.6,35 52.4,35.2 52.2,35.4 52,35.6 51.8,35.8 51.6,36 51.4,36.2 51.2,36.4 51,36.6 50.8,36.8 50.6,37 50.4,37.2 50.2,37.4 50,37.6 49.8,37.8 49.6,38 49.4,38.2 49.2,38.4 49,38.6 49,40.8 47,40.8 47,41 v46.2,41 | v44.4,42 39.4,42 38.6,42.8 36.8,42.8 36.6,43 36.4,43.2 36,43.2 35.8,43.4 35.6,43.6 35,44.2 34.8,44.4 34.4,44.4 33.6,45.2 v30.4,45.2
ECG_OPM  (via drill 0.3 pad 0.6)
  Top 0.2: 77.6,30.4 v77.6,30.2 | 80.4,31.6 80,32 78,32 77.8,31.8 77.6,31.6 | v77.8,26.4 78,26.4 78,27.8
  Bottom 0.2: v77.6,30.2 77.6,29.6 77.8,29.4 v78,29.2 | v77.6,23.2 77.6,26.2 v77.8,26.4
ECG_OPP  (via drill 0.3 pad 0.6)
  Top 0.2: 71.4,29.4 71.2,29.2 71.4,29.4 | 71.4,29.4 71.4,29.6 | 71.4,29.6 75.6,29.6 | 75.6,29.6 75.6,29.4 | 75.6,29.4 75.8,29.2 75.6,29.4 | 71.4,29.4 71.4,29.6 | 71.4,29.6 75.6,29.6 | 75.6,29.6 75.6,29.4
  Bottom 0.2: v78.4,23.2 78.4,26.4 78,26.8 77.8,27 77.6,27.2 v77,27.8
ECG_OUT
  Top 0.2: 85.8,34.2 85.8,35.2 | 88.2,31.6 88.2,32.4 88.6,32.8 88.8,33 89.6,33 89.8,33.2 90,33.4 90,35.6 86.2,35.6 | 29.8,61 43,61 43.2,60.8 43.6,60.4 53.2,60.4 53.4,60.2 53.6,60 53.8,59.8 54,59.6 54.2,59.4 54.4,59.2 54.6,59 54.8,58.8 55,58.6 55.2,58.4 55.4,58.2 55.6,58.2 55.8,58 57.2,58 57.4,57.8 57.6,57.6 57.8,57.4 58,57.2 60.6,57.2 61.2,56.6 61.4,56.4 61.6,56.2 62.2,55.6 62.4,55.4 62.6,55.2 63.2,54.6 63.4,54.4 63.6,54.2 64.2,53.6 64.4,53.4 64.6,53.2 64.8,53 65,52.8 65.2,52.6 65.4,52.4 65.6,52.2 65.8,52 66,51.8 66.2,51.6 66.4,51.4 66.6,51.2 66.8,51 67,50.8 67.2,50.6 67.4,50.4 67.6,50.2 67.8,50 68,49.8 68.2,49.6 68.4,49.4 68.6,49.2 68.8,49 72.6,49 72.8,48.8 73,48.6 73.2,48.4 73.6,48 73.8,47.8 74,47.6 74.2,47.4 74.6,47 74.8,46.8 75,46.6 75.2,46.4 75.6,46 75.8,45.8 76,45.6 76.2,45.4 76.6,45 76.8,44.8 77,44.6 77.2,44.4 77.6,44 77.8,43.8 78,43.6 78.2,43.4 78.6,43 78.8,42.8 79,42.6 79.2,42.4 79.6,42 79.8,41.8 80,41.6 80.2,41.4 80.6,41 80.8,40.8 81,40.6 81.2,40.4 81.6,40 81.8,39.8 82,39.6 82.2,39.4 82.6,39 82.8,38.8 83,38.6 83.2,38.4 83.6,38 83.8,37.8 84,37.6 84.2,37.4 84.4,37.2 84.6,37 84.8,36.8
  Top 0.25: U3.39 29.65,61.24
ECG_OUT_RAW  (via drill 0.3 pad 0.6)
  Top 0.15: U7.10 77,23.45 75.5,25.7
  Top 0.2: 83.6,32.4 83.6,31.6 83.6,32.4 | 83.6,32.4 83.8,32.6 | 83.8,32.6 84,32.8 83.8,32.6 | 79.8,30.2 79.6,30.4 79.8,30.2 | 79.8,30.2 80,30 | 80,30 82,30 | 82,30 82.2,30.2 | 82.2,30.2 82.4,30.4 82.2,30.2 | 83.6,32.4 83.8,32.6 | 79.8,30.2 80,30 | 80,30 82,30 | 82,30 82.2,30.2 | 75.8,25.8 76,26 76.2,26.2 v76.4,26.4 | v77.2,27 77.4,27.2 77.6,27.2 77.6,29.6 77.8,29.8 78,30 78.2,30.2 78.4,30.4
  Bottom 0.2: v76.4,26.4 76.8,26.8 77,27 v77.2,27
ECG_RA  (via drill 0.3 pad 0.6)
  Top 0.2: 85.8,21.2 v86,21.2
  Bottom 0.2: v86,21.2 96.4,21.2
ECG_RA_F
  Top 0.15: U7.3 80.45,21 82.7,21
  Top 0.2: 90.6,21.2 90.4,21 90.2,20.8 88.2,20.8 88,21 87.8,21.2 | 83,20.8 85,20.8 85.2,20.6 86.6,20.6 86.6,21.2
ECG_REFIN  (via drill 0.3 pad 0.6)
  Top 0.15: U7.18 78,18.55 78,16.3
  Top 0.2: 70.8,13.2 70.8,15.6 70.8,13.2 | 70.8,13.2 70.6,13 | 70.6,13 70.2,12.6 | 70.2,12.6 69.6,12.6 70.2,12.6 | 70.8,13.2 70.6,13 | 70.6,13 70.2,12.6 | 77.8,16.2 v76,16.2 | 70.4,11.4 69.6,11.4 70.4,11.4
  Bottom 0.2: v76,16.2 v71.2,16.2
ECG_REFOUT
  Top 0.15: U7.8 78,23.45 78,25.7
  Top 0.2: 81,29.2 82.8,29.2 83,29.4 83.2,29.6 83.8,29.6 84,29.8 84.2,30 84.4,30.2 84.8,30.6 85,30.8 85.2,31 85.4,31.2 85.8,31.6 86,31.8 86.2,32 86.4,32.2 86.6,32.4 87.4,32.4 87.4,33.2 87.6,33.4 87.8,33.6 88,33.8 | 78.2,25.8 78.2,26 78.4,26.2 78.8,26.6 79,26.8 79.2,27 79.4,27.2 79.6,27.4 79.6,27.6 79.8,27.8 | 73,27.8 73.2,27.8 73.6,27.4 76.2,27.4 76.4,27.2 76.6,27 76.8,26.8 77,26.6 77.4,26.2 77.6,26 77.8,25.8 | 73,9.2 72.8,9.4 72.6,9.6 72.2,10 72,10 72,27.8
ECG_RL  (via drill 0.3 pad 0.6)
  Top 0.2: 87.8,26.6 v88,26.6
  Bottom 0.2: v88,26.6 93.8,26.6 94,26.4 94.2,26.2 94.4,26 94.8,25.6 95,25.4 95.2,25.2 95.4,25 95.8,24.6 96,24.4 96.2,24.2 96.4,24
ECG_RLD
  Top 0.15: U7.5 80.45,22 82.7,23.5
  Top 0.2: 83,23.8 83,24.2 83.8,25 84,25.2 84.4,25.6 87.8,25.6 88,25.8 88.2,26 88.2,26.2 88.6,26.6 90,26.6 90.4,26.2 90.6,26 90.8,25.8 91,25.6 92.2,25.6 92.2,20.8 91,20.8 90.8,20.6 90.6,20.4 89,20.4 88.8,20.2 88.6,20 88,19.4 87.8,19.2 87.6,19 87,18.4 86.8,18.2 86,17.4 85.8,17.2 | 84.8,26.4 84.8,25.6
ECG_RLDFB  (via drill 0.3 pad 0.6)
  Top 0.2: v93,21.6 v93,20.8
  Bottom 0.2: v80.2,21.6 83.2,21.6 83.6,22 83.8,22.2 84,22.4 84.6,23 84.8,23.2 85,23.4 85.6,24 85.8,24.2 86,24.4 87.2,24.4 87.2,22.6 87.6,22.2 87.8,22 88,21.8 92.6,21.8 92.8,21.6 v93,21.6 | v93,20.8 91.4,20.8 91,20.4 90.8,20.2 90.6,20 90,19.4 89.8,19.2 89.6,19 89,18.4 88.8,18.2 88,17.4 v87.8,17.2
ECG_SDN  (via drill 0.3 pad 0.6)
  Top 0.15: U7.13 75.55,21 73.3,21
  Top 0.2: 73,21.2 v72.4,21.2 | v70.4,21.2 70.2,21.4 | 29.8,49.6 v31.8,49.6 | v33.8,49.6 41.8,49.6 46.2,45.2 49.6,45.2 49.6,45 49.8,44.8 50,44.6 50.2,44.4 50.4,44.2 50.6,44 50.8,43.8 51,43.6 51.2,43.4 51.4,43.2 51.6,43 51.8,42.8 52,42.6 52.2,42.4 52.4,42.2 52.6,42 52.8,41.8 53,41.6 53.2,41.4 53.4,41.2 53.6,41 53.8,40.8 v54,40.6 | v57.6,35.6 58,35.2 58.8,35.2 58.8,35 59.6,34.2 59.6,33.8 59.8,33.6 60.2,33.6 60.2,33 60.4,32.8 60.6,32.6 61.2,32 61.4,31.8 61.6,31.6 61.6,30.8 61.8,30.6 62,30.4 62.2,30.2 62.4,30 62.6,29.8 62.8,29.6 63,29.4 63.2,29.2 63.4,29 63.6,28.8 63.8,28.6 64,28.4 64.2,28.2 64.4,28 64.6,27.8 64.8,27.6 65.2,27.2 65.2,26.2 65.4,26 65.6,25.8 65.8,25.6 66.2,25.2 66.4,25 66.6,24.8 66.8,24.6 67.2,24.2 67.4,24 67.6,23.8 67.8,23.6 68.2,23.2 68.4,23 68.6,22.8 68.8,22.6
  Top 0.25: U3.30 29.65,49.81
  Bottom 0.2: v72.4,21.2 v70.4,21.2 | v31.8,49.6 v33.8,49.6 | v54,40.6 54,39.2 54.2,39 54.4,38.8 54.6,38.6 54.8,38.4 55,38.2 55.2,38 55.4,37.8 55.6,37.6 56.2,37 56.4,36.8 56.6,36.6 57.2,36 57.4,35.8 v57.6,35.6
ECG_SW  (via drill 0.3 pad 0.6)
  Top 0.15: U7.6 79,23.45 80.5,25.7
  Top 0.2: 82.2,10.2 82.4,10.4 82.2,10.2 | 82.2,10.2 82,10 | 82,10 81.8,9.8 | 81.8,9.8 81.6,9.6 | 81.6,9.6 81.4,9.4 | 81.4,9.4 81.2,9.2 | 81.2,9.2 81,9 | 81,9 80.8,8.8 | 80.8,8.8 80.6,8.6 | 80.6,8.6 80.4,8.4 | 80.4,8.4 80.4,7.4 | 80.4,7.4 76.4,7.4 | 76.4,7.4 76,7.8 76.4,7.4 | 80.6,25.8 82.2,25.8 82.4,26 82.6,26.2 82.8,26.4 83,26.6 83.4,27 83.6,27.2 83.8,27.4 84,27.6 84.4,28 88.2,28 88.8,27.4 89,27.2 89.2,27 90.4,27 90.8,26.6 91,26.4 91.2,26.2 91.4,26 92.6,26 92.6,20.4 92.4,20.2 92.2,20 92,19.8 91.8,19.6 91.4,19.2 91.2,19 91,18.8 90.8,18.6 90.6,18.4 90.4,18.2 90,17.8 89.8,17.6 89.6,17.4 89.4,17.2 89,16.8 88.8,16.6 88.6,16.4 88.4,16.2 88.2,16 88.2,15.4 87.4,15.4 87.2,15.2 87,15 86.8,14.8 86.6,14.6 86.4,14.4 86.2,14.2 86,14 85.8,13.8 85.6,13.6 85.4,13.4 85.2,13.2 85,13 84.8,12.8 84.6,12.6 84.4,12.4 84.2,12.2 84,12 83.8,11.8 83.6,11.6 | 82.2,10.2 82,10 | 82,10 81.8,9.8 | 81.8,9.8 81.6,9.6 | 81.6,9.6 81.4,9.4 | 81.4,9.4 81.2,9.2 | 81.2,9.2 81,9 | 81,9 80.8,8.8 | 80.8,8.8 80.6,8.6 | 80.6,8.6 80.4,8.4 | 80.4,8.4 80.4,7.4 | 80.4,7.4 76.4,7.4 | 75.2,28.4 v75.4,28.4
  Bottom 0.2: v79.2,22.4 79.4,22.4 79.4,14.6 79.6,14.4 79.8,14.2 80,14 80.4,13.6 80.6,13.4 80.8,13.2 81,13 81.4,12.6 81.6,12.4 81.8,12.2 82,12 v82.4,11.6 | v75.4,28.4 77.6,28.4 77.8,28.2 78,28 78.8,27.2 79,27 79.8,26.2 80,26 v80.2,25.8
ESP_EN
  Top 0.25: U3.3 4.95,59.97
ESP_IO0  (via drill 0.3 pad 0.6)
  Top 0.2: v33.6,51.6 33.8,51.6 33.8,56.4 35.8,58.4 | 28.4,46.4 v28.6,46.4
  Top 0.25: U3.27 27.75,42.4
  Bottom 0.2: v34.2,48 34.2,50.8 34,51 33.8,51.2 33.6,51.4 v33.6,51.6 | v28.6,46.4 32.2,46.4 32.6,46.8 32.8,47 33,47.2 33.6,47.8 33.8,48 34,48.2 34.2,48.2 | 2.8,37.2 3,37.4 3.4,37.8 3.6,38 3.8,38.2 4,38.4 4.2,38.6 4.4,38.8 4.6,39 4.8,39.2 5,39.4 5.2,39.6 5.4,39.8 5.6,40 5.8,40.2 6,40.4 6.2,40.6 6.4,40.8 6.6,41 6.8,41.2 7,41.4 7.2,41.6 7.4,41.8 7.6,42 7.8,42.2 8,42.4 8.2,42.6 8.4,42.8 8.4,59.2 10.2,59.2 10.4,59.4 10.6,59.6 12,59.6 12.2,59.4 12.4,59.2 12.6,59 12.8,58.8 13,58.6 13.2,58.4 13.4,58.2 13.6,58 13.8,57.8 14,57.6 14.2,57.4 14.4,57.2 14.6,57 14.8,56.8 15,56.6 15.2,56.4 15.4,56.2 15.6,56 15.8,55.8 16,55.6 16,53 19,53 19.2,52.8 19.4,52.6 19.6,52.4 20,52 20.2,51.8 20.4,51.6 20.6,51.4 21,51 21.2,50.8 23,50.8 23.2,50.6 23.4,50.4 23.8,50 24,49.8 24.2,49.6 24.4,49.4 24.8,49 25,48.8 25.2,48.6 25.4,48.4 25.8,48 26,47.8 26.2,47.6 26.4,47.4 26.8,47 27,46.8 27.2,46.6 v27.2,46.4
FSR1_ADC  (via drill 0.3 pad 0.6)
  Top 0.2: 33.6,10.6 34.6,10.6 34.8,10.8 | 37.2,9.4 37,9.4 36.8,9.6 36.4,10 36.2,10.2 36,10.4 | v20,27.4 20,27 v19.6,26.6 | v30,11 31.8,11 32,10.8 32.2,10.6
  Top 0.25: U3.4 6.65,58.7
  Bottom 0.2: v9.6,58.2 9.6,42.4 10,42 10.2,41.8 10.4,41.6 10.6,41.4 11,41 11.2,40.8 11.2,38.4 11.4,38.2 11.6,38 11.6,37.8 12,37.4 12.2,37.2 12.4,37 12.6,36.8 13,36.4 13.2,36.2 13.4,36 13.6,35.8 14,35.4 14.2,35.2 14.4,35 14.6,34.8 15,34.4 15.2,34.2 15.4,34 15.6,33.8 16,33.4 16.2,33.2 16.4,33 16.6,32.8 17,32.4 17.2,32.2 19,30.4 19.2,30.2 19.4,30 19.4,28.2 19.6,28 20,27.6 v20,27.4 | v19.6,26.6 19.6,24 20,23.6 20.2,23.4 20.4,23.2 20.6,23 21,22.6 21.2,22.4 21.2,20.8 21.4,20.6 21.4,20.2 21.6,20 21.6,19.4 21.8,19.2 22,19 22.2,18.8 22.6,18.4 22.8,18.2 23,18 23.2,17.8 23.6,17.4 23.8,17.2 23.8,17 24,16.8 24.2,16.6 24.4,16.4 24.6,16.2 25,15.8 25.2,15.6 25.4,15.4 25.6,15.2 25.8,15 26,14.8 26.2,14.6 26.4,14.4 26.6,14.2 26.8,14 27,13.8 27.2,13.6 27.4,13.4 27.6,13.2 27.8,13 28,12.8 28.2,12.6 28.4,12.4 28.6,12.2 28.8,12 29,11.8 29.2,11.6 29.4,11.4 29.6,11.2 29.8,11 v30,11
FSR2_ADC  (via drill 0.3 pad 0.6)
  Top 0.2: 40.2,9.4 40,9.6 39.8,9.8 39.8,11.6 39.6,11.8 39.4,12 39.2,12.2 39.2,13.6 39,13.8 38.8,14 38.6,14.2 38.4,14.4 38.2,14.6 38,14.8 37.8,15 37.6,15.2 v37.6,17 | 42.8,8.2 42.6,8 41.6,8 41.6,8.2
  Top 0.25: U3.5 8.35,57.43
  Bottom 0.2: v37.6,17 37.6,17.2 36.4,17.2 | v10.2,57 10.2,42.6 10.4,42.4 10.6,42.2 10.8,42 11,41.8 11.2,41.6 11.4,41.4 11.6,41.2 11.8,41 12,40.8 12.2,40.6 12.4,40.4 12.6,40.2 12.8,40 13,39.8 13.2,39.6 13.4,39.4 13.6,39.2 13.8,39 14,38.8 14.2,38.6 14.4,38.4 14.6,38.2 14.8,38 15,37.8 15.2,37.6 15.4,37.4 15.6,37.2 15.8,37 16,36.8 16.2,36.6 16.4,36.4 16.6,36.2 16.8,36 17,35.8 17.2,35.6 17.4,35.4 17.6,35.2 17.8,35 18,34.8 18.2,34.6 18.4,34.4 18.6,34.2 18.8,34 19,33.8 19.2,33.6 19.4,33.4 19.6,33.2 19.8,33 20,32.8 20.2,32.6 20.4,32.4 20.6,32.2 20.8,32 21,31.8 21.2,31.6 21.6,31.2 21.8,31 22,30.8 22.2,30.6 22.6,30.2 22.8,30 23,29.8 23.2,29.6 23.6,29.2 23.8,29 24,28.8 24.2,28.6 24.6,28.2 24.8,28 24.8,26.8 26,26.8 26.2,26.6 26.6,26.2 26.8,26 27,25.8 27.2,25.6 27.6,25.2 27.8,25 28,24.8 28,24.2 31.4,20.8 32,20.8 32.2,20.6 32.4,20.4 32.6,20.2 32.8,20 33,19.8 33.2,19.6 33.4,19.4 33.6,19.4 33.6,19.2 33.8,19 34,18.8 34.2,18.6 34.4,18.4 34.6,18.2 34.8,18 35,17.8
FSR3_ADC  (via drill 0.3 pad 0.6)
  Top 0.2: 51,14.2 50.8,14.2 50.6,14.4 50.4,14.6 50,15 49.8,15.2 49.6,15.4 49.6,17.8 48.8,17.8 48.6,18 47,18 46.8,18.2 42.4,18.2 42.2,18.4 42,18.6 41.8,18.8 41.6,19 v41.4,19.2 | 49.6,9.4 49.8,9.6 50,9.8 50,12 50.2,12.2 50.4,12.4 50.6,12.6 50.8,12.8 51,13 | 11,55.8 11.4,55.8 11.4,55.4 11.6,55.2 v11.6,52.4 | v11.6,48.4 v11.6,46 | v28.4,29 28.4,28.4 28.6,28.4 28.8,28.2 29,28 29.2,27.8 29.8,27.2 30,27 30.2,26.8 30.8,26.2 31,26 31.2,25.8 31.8,25.2 31.8,25 34,25 34,24.8 34.2,24.6 34.4,24.4 34.6,24.2 34.8,24 35,23.8
  Bottom 0.2: v41.4,19.2 40,19.2 39.8,19.4 39.6,19.6 39.4,19.8 39.2,20 39,20.2 38.8,20.4 38.6,20.6 38.4,20.8 38.2,21 38,21.2 37.8,21.4 37.4,21.8 37.2,22 37,22.2 36.8,22.4 36.4,22.8 | v11.6,52.4 v11.6,48.4 | v11.6,46 11.6,44.8 11.8,44.6 12,44.4 12.2,44.2 12.4,44 12.6,43.8 12.8,43.6 13,43.4 13.2,43.2 13.4,43 13.6,42.8 13.8,42.6 14,42.4 14.2,42.2 14.4,42 14.6,41.8 14.8,41.6 15,41.4 15.2,41.2 15.4,41 15.6,40.8 15.8,40.6 16,40.4 16.2,40.2 16.4,40 16.6,39.8 16.8,39.6 17,39.4 17.2,39.2 17.4,39.2 17.6,39 17.8,38.8 18,38.6 18.2,38.4 18.4,38.2 18.6,38 18.8,37.8 19,37.6 19.2,37.4 19.4,37.2 19.6,37 19.8,36.8 20,36.6 20.2,36.4 20.4,36.2 20.6,36 20.8,35.8 21,35.6 21.2,35.4 21.4,35.2 21.6,35 21.8,34.8 22,34.6 22.2,34.4 22.4,34.2 22.6,34 22.8,33.8 23,33.6 23.2,33.4 23.4,33.2 23.6,33 23.8,32.8 24.8,32.8 25,32.6 25.2,32.4 25.4,32.2 25.6,32 26,31.6 26.2,31.4 26.4,31.2 26.6,31 27,30.6 27.2,30.4 27.4,30.2 27.6,30 28,29.6 28.2,29.4 28.4,29.2 v28.4,29
FSR4_ADC  (via drill 0.3 pad 0.6)
  Top 0.2: 53.8,14.2 v52.8,14.2 | v43.6,20 43.4,20.2 43,20.6 42.8,20.8 42.6,21 42.4,21.2 42,21.6 41.8,21.8 41.6,22 v41.4,22.2 | 51.8,7.6 51.6,7.8 51.4,8 51.4,11.8 51.6,12 51.8,12.2 52,12.4 52.2,12.6 52.8,12.6 53,12.8 53.2,13 53.8,13 | v32.8,32.4 33.2,32 33.4,31.8 33.8,31.4 34,31.2 34.2,31 34.4,30.8 34.8,30.4 35,30.2 35.2,30
  Bottom 0.2: v52.8,14.2 50.6,14.2 50.4,14.4 50.2,14.6 50,14.8 49.8,15 49.6,15.2 49.4,15.4 49.2,15.6 49,15.8 48.8,16 48.6,16.2 48.4,16.4 48,16.8 47.8,17 47.6,17.2 47.4,17.4 47,17.8 46.8,18 46.6,18.2 46.4,18.4 46,18.8 45.8,19 45.6,19.2 45.4,19.4 45,19.8 44.8,20 v43.6,20 | v41.4,22.2 41,22.6 40.8,22.8 40.6,23 40.4,23.2 40,23.6 39.8,23.8 39.6,24 39.6,24.8 39.4,25 39.2,25.2 39,25.4 38.8,25.6 38.6,25.8 38.4,26 38.2,26.2 38,26.4 37.8,26.6 37.4,27 37.2,27.2 37,27.4 36.8,27.6 36.4,28 36.2,28.2 36,28.4 | v11,54.4 11,54.2 11.2,54 11.4,53.8 11.6,53.6 11.8,53.4 12,53.2 12.2,53 12.4,52.8 12.6,52.6 12.8,52.4 13,52.2 13.2,52 13.4,51.8 13.6,51.6 13.8,51.4 14,51.2 14.2,51 14.4,50.8 14.6,50.6 14.8,50.4 15,50.2 15.2,50 15.4,49.8 15.6,49.6 15.8,49.4 16.2,49 16.4,48.8 16.6,48.6 16.8,48.4 17.2,48 17.4,47.8 17.6,47.6 17.8,47.4 18.2,47 18.4,46.8 18.6,46.6 18.8,46.4 19,46.2 19.2,46 19.4,45.8 19.6,45.6 19.8,45.4 20,45.2 20.2,45 20.4,44.8 20.6,44.6 20.8,44.4 21,44.2 21.2,44 21.4,43.8 21.6,43.6 21.8,43.4 22,43.2 22.2,43 22.4,42.8 22.6,42.6 22.8,42.4 23,42.2 23.2,42 23.4,41.8 23.6,41.6 23.8,41.4 24,41.2 24.2,41 24.4,40.8 24.6,40.6 24.8,40.4 25,40.2 25.2,40 25.4,39.8 25.6,39.6 25.8,39.4 26,39.2 26.2,39 26.4,38.8 26.6,38.6 26.8,38.4 27,38.2 27.2,38 27.4,37.8 27.8,37.4 28,37.2 28.2,37 28.4,36.8 28.8,36.4 29,36.2 29.2,36 29.4,35.8 29.8,35.4 30,35.2 30.2,35 30.4,34.8 30.8,34.4 31,34.2 31.2,34 31.4,33.8 31.8,33.4 32,33.2 v32.8,32.4
GND  (via drill 0.3 pad 0.55, 0.3 pad 0.6)
  Top 0.15: U5.3 44.7,38.75 47.65,38.42 | U5.2 44.7,39.25 46.4,39.58 | U5.1 44.7,39.75 47.65,40.73 | U5.7 42.5,37.3 41.85,35.6 | U5.6 43,37.3 43,34.35 | U7.16 77,18.55 75.5,16.3
  Top 0.2: U4.2 51,39.5 48.4,39.5 | U4.4 54,38.85 55.4,38.35 | U8.5 38.8,18.86 35.3,18.8 | U8.4 38.8,20.14 36.8,20.2 | U8.10 45.7,15.3 | 45.7,15.3 43.7,13.3 | U8.9 45.7,15.3 | 45.7,15.3 45.1,11.8 | U8.14 47.2,21.41 50.7,21.6
  Top 0.25: U1.1 15.4,16.91 | U1.3 15.4,14.37 | U3.1 6.65,62.51 | U3.40 31.35,62.51 | U6.4 45.4,32.09 | U6.8 54.6,35.91
  Top 0.3: 15.4,16.91 v15.4,17.61 | 15.4,14.37 v15.4,13.66 | R1.2 v25.45,11.9 | C1.2 v13,15.22 | C2.2 v16.4,29.95 | U2.2 v11,19.45 | C3.2 v14.5,19.23 | C4.2 v20.4,20.7 | C5.2 v23.4,20.7 | R6.2 v23.6,24.95 | C6.2 v27.5,28.73 | TP3.TP v24.5,33.45 | 6.65,62.51 v6.65,61.81 | 31.35,62.51 v31.35,63.21 | C7.2 v5.2,62.45 | C8.2 v5.2,58.45 | C10.2 v4.8,53.23 | D3.1 v43.27,59 | D4.1 v44.55,52.6 | 48.4,39.5 v48.4,40.2 | 55.4,38.35 v55.4,39.05 | C11.2 v48.5,47.48 | 47.65,40.73 v47.65,41.42 | 46.4,39.58 v46.4,40.27 | 47.65,38.42 v47.65,39.12 | 43,34.35 v43,35.05 | 41.85,35.6 v41.85,36.3 | C12.2 v38.9,36.45 | C13.2 v37.5,41.73 | 45.4,32.09 v45.4,32.8 | 54.6,35.91 v54.6,36.6 | C14.2 v44.75,33.73 | C15.2 v55.25,33.73 | U7.14 v77.35,20.5 | 75.5,16.3 v75.5,17 | R24.2 v74.22,11 | C16.2 v70.2,13.95 | C22.2 v89.45,32.4 | R32.2 v69.5,27.23 | C23.2 v75.95,14.9 | C24.2 v78.95,12.4 | 36.8,20.2 v37.5,20.2 | 35.3,18.8 v36,18.8 | 45.1,11.8 v45.1,12.5 | 43.7,13.3 v43.7,14 | 50.7,21.6 v50.7,22.3 | U8.15 v45.7,21.68 | C25.2 v33,17.23 | C26.2 v34.4,21.95 | C27.2 v50.35,21.95 | C28.2 v33,27.23 | R33.2 v31.6,11.95 | C29.2 v38,11.97 | R34.2 v41,11.97 | C30.2 v43.5,11.97 | R35.2 v49,11.97 | C31.2 v53.15,15.45 | R36.2 v53.9,8.95 | C32.2 v55.9,15.45 | R37.2 v59.4,11.45 | C33.2 v55.6,15.45 | R38.2 v56.4,8.95 | R40.2 v56.75,20.73 | C35.2 v60.9,16.95 | D6.2 v54,25.55 | C36.2 v46.5,11.97 | Q1.2 v75.95,59.05 | R44.2 v71.4,56.45 | C37.2 v75,66.22 | Q2.2 v75.95,54.55 | R47.2 v71.4,49.95 | C38.2 v79,53.73 | C39.2 v53.5,58.23
  other vias: 16.65,53.65 16.65,54.75 16.65,55.85 17.75,53.65 17.75,54.75 17.75,55.85 18.85,53.65 18.85,54.75 18.85,55.85 52.5,39.95 52.5,39.05 78.7,21.7 77.3,21.7 78.7,20.3 77.3,20.3 7,7 7,18 7,29 7,40 7,62 18,7 18,18 18,29 18,40 18,51 18,62 29,7 29,18 29,29 29,40 29,62 40,7 40,29 40,40 40,51 40,62 51,7 51,29 51,62 62,7 62,18 62,29 62,51 62,62 73,7 73,18 73,40 73,51 73,62 84,7 84,18 84,29 84,40 84,51 84,62
  pour Route2 (isolate 0.4): 0.5,0.5 99.5,0.5 99.5,69.5 29.5,69.5 29.5,63 0.5,63
HALL_LIMIT  (via drill 0.3 pad 0.6)
  Top 0.2: 47.2,8.2 47.2,4.6 47.4,4.4 47.6,4.2 47.8,4 48,3.8 | 33.6,7.4 38,7.4 38.4,7 38.6,6.8 38.8,6.6 39,6.4 39.2,6.2 43.8,6.2 44,6.4 44.4,6.8 44.6,7 44.8,7.2 45,7.4 45.4,7.8 45.6,8 45.8,8.2 | 27,55.2 25.2,55.2 25,55.4 24.4,55.4 24.2,55.6 24,55.8 23.8,56 v23.6,56.2 | v19.4,60.2 13,60.2 12.8,60.4 12.6,60.6 12.4,60.8 12.2,61 12,61.2 11.8,61.4 v11.6,61.6 | v5.8,41 5.8,39.6 6,39.4 6.4,39 6.6,38.8 6.8,38.6 7,38.4 7.4,38 7.6,37.8 7.8,37.6 8,37.4 8.2,37.2 8.4,37 8.6,36.8 8.8,36.6 9,36.4 9.2,36.2 9.4,36 9.6,35.8 10,35.4 10.2,35.2 10.4,35 10.6,34.8 11,34.4 11.2,34.2 11.4,34 11.6,33.8 12,33.4 12.2,33.2 12.4,33 v12.6,32.8
  Top 0.25: U3.34 31.35,54.89
  Bottom 0.2: v23.6,56.2 23.4,56.4 23.2,56.6 23,56.8 22.8,57 22.4,57.4 22.2,57.6 22,57.8 21.8,58 21.4,58.4 21.2,58.6 21,58.8 20.8,59 20.4,59.4 20.2,59.6 20,59.8 19.8,60 19.6,60.2 v19.4,60.2 | v11.6,61.6 10.2,61.6 10,61.8 9.8,62 9.6,62.2 9.4,62.4 9.2,62.6 9,62.8 6.4,62.8 6.2,63 6,63.2 5.8,63.4 4.6,63.4 4.4,63.2 4.4,56.2 4.6,56 4.6,54.6 4.4,54.4 4,54 4,52.2 4.2,52 4.4,51.8 4.6,51.6 4.8,51.4 5,51.2 5.2,51 5.4,50.8 5.6,50.6 5.8,50.4 6,50.2 6.2,50 6.2,42.8 6,42.6 5.8,42.4 v5.8,41 | v12.6,32.8 13,32.4 13.2,32.2 13.4,32 14.4,32 14.6,31.8 16.8,31.8 17.2,31.4 17.4,31.2 17.6,31 18.2,30.4 18.4,30.2 18.6,30 19,29.6 19,27.8 19.2,27.6 19.6,27.2 19.8,27 20,26.8 20.2,26.6 20.6,26.2 20.8,26 21,25.8 21.2,25.6 21.2,25.4 21.4,25.2 21.6,25 22,24.6 22.2,24.4 22.4,24.2 22.6,24 23,23.6 23.2,23.4 23.4,23.2 23.4,22.2 23.6,22 24,21.6 24.2,21.4 24.2,17.4 24.4,17.2 25,16.6 25.2,16.4 25.4,16.2 26,15.6 26.2,15.4 26.4,15.2 26.6,15 27,14.6 27.2,14.4 27.4,14.2 27.6,14 28,13.6 28.2,13.4 28.4,13.2 28.6,13 29,12.6 29.2,12.4 29.4,12.2 29.6,12 30,11.6 30.2,11.4 30.4,11.2 30.6,11 31,10.6 31.2,10.4 31.4,10.2 31.6,10 32,9.6 32.2,9.4 v32.2,8.6
HX_BASE  (via drill 0.3 pad 0.6)
  Top 0.2: 39.6,22.4 v39.6,22.2 | v42,20 42.4,19.6 42.6,19.4 42.8,19.2 v44.2,19.2
  Bottom 0.2: v39.6,22.2 39.6,22 39.8,21.8 40,21.6 40.4,21.2 40.8,21.2 41,21 41.4,20.6 41.6,20.4 41.8,20.2 v42,20 | v44.2,19.2 44.8,19.2 45,19 45.4,18.6 45.6,18.4 45.8,18.2 46,18 46.4,17.6 46.6,17.4 46.8,17.2 47,17 47.4,16.6 47.6,16.4 47.8,16.2 48,16 48.4,15.6 48.6,15.4 48.8,15.2 49,15 49.4,14.6 49.6,14.4 49.8,14.2 50,14 50.2,13.8 51.8,13.8 52,13.6 56.8,13.6 56.8,14.8 56.6,15 56.6,16.2 56.4,16.4 56,16.8 56,17.4 v52.4,17.4
HX_DOUT  (via drill 0.3 pad 0.6)
  Top 0.2: U8.12 47.2,18.86 50.7,18.8 | 51,19 52.8,19 52.8,20 53,20.2 53.4,20.6 53.6,20.8 54.6,20.8 54.8,21 55,21.2 55.6,21.2 55.6,23.2 | 22.4,42.6 22.6,42.4 v22.6,39.6 | v23.4,33.8 v23.4,32.4 | v23.8,29.6 v23.8,28.4 | v24.4,26 23.4,26 23.2,25.8 23,25.6 v23,24.4 | v23.8,23.6 24,23.4 24,22 27.6,22 27.8,22.2 28,22.4 28.2,22.6 28.6,23 28.8,23.2 29,23.4 v29.2,23.6 | v46.8,16.6 46.8,17.2 47.6,17.2 47.8,17 v48.4,17 | v47.4,18.4 47.2,18.6 46.4,18.6
  Top 0.25: U3.23 22.18,42.85
  Bottom 0.2: v22.6,39.6 22.6,39.4 23,39 23.2,38.8 23.4,38.6 v23.4,33.8 | v23.4,32.4 23.6,32.2 23.8,32 v23.8,29.6 | v23.8,28.4 23.8,28.2 24,28 24.2,27.8 24.4,27.6 v24.4,26 | v23,24.4 23,24.2 23.2,24.2 23.4,24 v23.8,23.6 | v29.2,23.6 29.4,23.6 29.8,23.2 30,23 30.2,22.8 30.8,22.2 31,22 31.2,21.8 31.2,21.6 32.8,21.6 33,21.4 33.2,21.2 33.4,21 33.8,20.6 34,20.4 34.2,20.2 34.4,20 34.8,19.6 38.8,19.6 39,19.4 39.2,19.2 39.4,19 39.6,18.8 40.4,18.8 40.6,18.6 40.8,18.4 42.8,18.4 43,18.2 43.2,18 43.6,18 43.8,17.8 44,17.6 44.2,17.4 44.4,17.2 46,17.2 46.4,16.8 46.6,16.6 v46.8,16.6 | v48.4,17 48.4,17.4 48,17.8 47.8,18 47.6,18.2 v47.4,18.4
HX_SCK  (via drill 0.3 pad 0.6)
  Top 0.2: U8.11 47.2,17.59 49.2,17.4 | v42.8,21.6 42.8,23.8 v42.6,24 | v41.8,27.8 41.8,28.4 41.6,28.6 41.4,28.8 41.2,29 41,29.2 40.8,29.4 40.6,29.6 39.8,29.6 39.8,30.2 39.6,30.4 39.4,30.6 v39.2,30.8 | v35.8,33.4 35,34.2 34.6,34.2 34.6,34.6 v34.4,34.8 | v33.8,35.6 33.8,39.6 33.6,39.8 33.4,40 33.2,40.2 32.6,40.8 32.4,41 v32.2,41.2 | v30.4,43 30.2,43.2 30,43.4 29.8,43.6 29.6,43.8 29.4,44 29.2,44.2 29,44.4 28.8,44.6 28.6,44.8 28.4,45 v28.2,45.2 | v26,47.2 v26,48.4 | v26.4,50 26.6,50.2 26.6,50.6 27,50.6
  Top 0.25: U3.31 31.35,51.08
  Bottom 0.2: v45,17.8 44.8,18 44.6,18.2 44.4,18.4 43.6,18.4 43.4,18.6 43,19 42.8,19.2 v42.8,21.6 | v42.6,24 42.4,24.2 42.4,26.6 42,27 41.8,27.2 v41.8,27.8 | v39.2,30.8 39,31 38.8,31.2 38.6,31.4 38.4,31.6 38,32 37.8,32.2 37.6,32.4 37.4,32.6 37.2,32.8 37,33 36.8,33.2 36.6,33.4 v35.8,33.4 | v34.4,34.8 33.8,35.4 v33.8,35.6 | v32.2,41.2 32,41.4 31.8,41.6 31.6,41.8 31.4,42 31.2,42.2 31,42.4 30.8,42.6 30.6,42.8 v30.4,43 | v28.2,45.2 28,45.4 26,45.4 v26,47.2 | v26,48.4 26,49.6 26.2,49.8 v26.4,50
HX_VBG  (via drill 0.3 pad 0.6)
  Top 0.2: U8.6 38.8,17.59 36.8,17.4 | 36.8,17.2 v36.8,16.4
  Bottom 0.2: v36.8,16.4 36.6,16.2 36.4,16 34.8,16 34.4,15.6 34.4,15.4 34.2,15.2 34,15 33.8,14.8 v33.6,14.6
HX_XO  (via drill 0.3 pad 0.6)
  Top 0.2: U8.13 47.2,20.14 49.2,20.2 | 49,20.4 v49,21
  Bottom 0.2: v49,21 48.8,21.2 48.8,22.8 49.8,22.8 50,23 50.4,23 50.6,23.2 50.8,23.4 v51,23.6
I2C_SCL  (via drill 0.3 pad 0.6)
  Top 0.15: U5.13 43,40.7 43,43.65
  Top 0.2: U4.1 51,40.15 49.6,40.65 | 43.2,43.4 45.2,43.4 45.4,43.2 45.6,43 45.8,42.8 46,42.6 46.2,42.4 46.4,42.2 48.4,42.2 48.6,42 48.8,41.8 49,41.6 v52.4,41.6 | v59.4,45.4 60.6,46.6 v60.6,47.4 | v62.4,50.2 64.8,50.2 65,50.4 65.2,50.6 65.4,50.8 65.6,51 v65.8,51.2 | v66.6,39.6 66.4,39.4 66,39 65.8,38.8 65.6,38.6 65.6,29.2 65.4,29 v65.4,28.8 | v64.2,24.4 64,24.2 63.8,24 63.6,23.8 63.4,23.6 63,23.2 62.8,23 62.6,22.8 62.4,22.6 62,22.2 61.8,22 61.6,21.8 61.4,21.6 61,21.2 60.8,21 60.6,20.8 60.4,20.6 v60,20.2 | 49.4,40.8 49.4,41.6 | 58.8,51.2 v59,51.2 | 40.8,46.4 41,46.4 41.4,46 41.4,45.2 41.6,45 41.8,44.8 42,44.6 42.2,44.4 42.4,44.2 42.6,44 42.8,43.8 | 9.6,52.6 8.4,52.6 8.2,52.8 8,53 7.8,53.2 7.6,53.4 7.6,55 v7.4,55 | v41,65.2 42.6,65.2 42.8,65 43,65 43.2,64.8 43.4,64.6 43.6,64.4 43.8,64.2 44,64 44.2,63.8 44.8,63.2 47.8,63.2 48,63 48.2,62.8 48.8,62.2 v48.8,62 | v48,58 47.8,57.8 47.8,53 47.6,52.8 47.4,52.6 46,52.6 45.6,52.2 45.4,52 45.2,51.8 45,51.8 44.8,51.6 44.6,51.4 44.4,51.2 44.2,51 44,50.8 43.8,50.6 43.6,50.4 43.4,50.2 43.2,50 43,49.8 v42.8,49.6
  Bottom 0.2: v52.4,41.6 54.2,41.6 54.8,42.2 56.2,42.2 v59.4,45.4 | v60.6,47.4 60.6,48 60.8,48.2 60.8,48.6 61,48.8 61.2,49 | 61.2,49 61.4,49.2 61.6,49.4 61.8,49.6 62,49.8 62.2,50 v62.4,50.2 | v65.8,51.2 66,51.4 66.4,51.4 66.6,51.6 66.8,51.8 67,52 67.4,52.4 67.6,52.6 69.2,52.6 69.4,52.4 69.4,42.4 69,42 68.8,41.8 68.6,41.6 68.4,41.4 68,41 67.8,40.8 67.6,40.6 67.4,40.4 67,40 66.8,39.8 v66.6,39.6 | v65.4,28.8 65.4,25.6 65,25.2 64.8,25 64.6,24.8 v64.2,24.4 | v60,20.2 59.8,20 59.8,19.8 59.6,19.6 59.4,19.4 59.2,19.2 59,19 58.8,18.8 58.6,18.6 58.4,18.4 58.2,18.2 58.2,15.6 58,15.4 57.8,15.2 57.8,12.8 57.6,12.6 57.4,12.4 57.2,12.2 57.2,8.2 57,8 56.8,7.8 56.8,7.2 56.6,7 55.6,7 55.4,6.8 55.2,6.6 52,6.6 51.8,6.4 51.6,6.2 46.2,6.2 46,6 45.8,5.8 45.6,5.6 45.4,5.4 45,5 44.8,4.8 44.6,4.6 44.4,4.4 44,4 43.8,3.8 43.6,3.6 43.4,3.4 43,3 42.8,2.8 42.6,2.6 42.4,2.4 42,2 41.8,1.8 31.6,1.8 31.4,2 31.2,2.2 31,2.4 30.8,2.6 | v59,51.2 59.2,51.2 60.8,49.6 60.8,49.4 61,49.2 61.2,49 | v7.4,55 7.4,56.8 7.2,57 7,57.2 6.8,57.4 6.6,57.6 6.6,59.2 6.8,59.4 7,59.6 7,60.4 7.2,60.6 9,60.6 9.2,60.8 9.4,61 26.6,61 27,61.4 27.2,61.6 27.4,61.8 27.6,62 28,62.4 28.2,62.6 28.4,62.8 29.4,62.8 29.6,63 29.6,63.8 29.8,64 30,64.2 30.2,64.4 30.4,64.6 30.6,64.8 31,65.2 31.2,65.4 31.4,65.6 31.6,65.8 32,66.2 32.2,66.4 32.4,66.6 32.6,66.8 32.8,67 33,67.2 33.2,67.4 33.4,67.6 33.6,67.8 33.8,68 34,68.2 34.2,68.4 34.4,68.6 35.4,68.6 35.6,68.8 37,68.8 37.2,68.6 37.2,67.2 37.4,67 37.6,66.8 37.8,66.6 38,66.4 38.4,66 38.6,65.8 38.8,65.6 39,65.4 39.2,65.2 v41,65.2 | v48.8,62 48.8,60.2 48.6,60 48.6,59.8 48.4,59.6 48.4,58.4 v48,58
  Bottom 0.2: v42.8,49.6 42.6,49.4 42.4,49.2 42.2,49 42,48.8 41.8,48.6 41.6,48.4 41.4,48.2 41.2,48 41,47.8 v40.8,47.6
I2C_SDA
  Top 0.15: U5.14 43.5,40.7 44.15,42.4
  Top 0.2: U4.6 54,40.15 55.4,40.65
  Top 0.25: U3.8 8.35,53.62
IMU_INT1  (via drill 0.3 pad 0.6)
  Top 0.15: U5.4 44.7,38.25 46.4,37.27
  Top 0.2: 46.6,37 v46.6,36.6 | 11,50.6 17,50.6 17.2,50.4 17.6,50.4 18,50 18.2,49.8 18.4,49.6 18.6,49.4 v18.8,49.2 | v24.4,48.8 v26.6,48.8 | v28.8,48 29,47.8 29.2,47.6 29.4,47.4 29.8,47 30,46.8 30.2,46.6 30.4,46.4 v30.8,46 | v31.6,46 31.8,45.8 32,45.6 32.2,45.4 32.4,45.2 32.6,45 32.8,44.8 33,44.6 33.2,44.4 33.4,44.2 33.6,44 33.6,43.2 v33.8,43.2 | v40,37 40.2,36.8 40.4,36.6 40.6,36.4 40.8,36.2 41,36 41.2,35.8 41.2,35.6 41.4,35.4 41.4,35.2 41.6,35 41.8,34.8 42,34.6 42.2,34.4 42.4,34.2 42.6,34 42.8,33.8 42.8,33.2 43,33 43.2,32.8 43.4,32.6 43.6,32.4 43.6,29 43.8,28.8 44,28.6 45.4,28.6 45.6,28.8 45.8,29 46,29.2 46.8,29.2
  Top 0.25: U3.10 6.65,51.08
  Bottom 0.2: v46.6,36.6 47.2,36 47.4,35.8 47.6,35.6 48.2,35 48.4,34.8 48.6,34.6 49.2,34 49.2,31.8 49,31.6 48.8,31.4 48.6,31.2 48.4,31 v48.2,30.8 | v18.8,49.2 22.4,49.2 22.6,49 22.8,48.8 v24.4,48.8 | v26.6,48.8 28,48.8 28.2,48.6 28.4,48.4 v28.8,48 | v30.8,46 v31.6,46 | v33.8,43.2 34,43 34.2,42.8 34.4,42.6 34.6,42.4 34.8,42.2 35,42 35.2,41.8 36,41.8 36.8,41 38.8,41 39,40.8 40.4,40.8 40.6,40.6 40.6,37.8 40.4,37.6 40.2,37.4 40.2,37.2 40,37.2 v40,37
IMU_INT2  (via drill 0.3 pad 0.6)
  Top 0.15: U5.9 41.3,38.75
  Top 0.2: 41,38.8 40,38.8 v39.8,39 | v19.8,46 14.8,46 14.6,46.2 14.4,46.4 14.2,46.6 14,46.8 13.8,47 13.6,47.2 13.4,47.4 13.2,47.6 13,47.8 12.8,48 12.6,48.2 12.4,48.4 12.2,48.6 12,48.8 11.8,49 11.6,49.2 11.4,49.4 11,49.4
  Top 0.25: U3.11 8.35,49.81
  Bottom 0.2: v39.8,39 39.6,39.2 26.8,39.2 26.6,39.4 26.4,39.6 26.2,39.8 26,40 25.6,40.4 25.4,40.6 25.2,40.8 25,41 24.6,41.4 24.4,41.6 24.2,41.8 24,42 23.6,42.4 23.4,42.6 23.2,42.8 23,43 22.6,43.4 22.4,43.6 22.2,43.8 22,44 21.6,44.4 21.4,44.6 21.2,44.8 21,45 20.6,45.4 20.4,45.6 20.2,45.8 20,46 v19.8,46
IMU_OCS_AUX
  Top 0.15: U5.10 41.3,39.25 39.6,39.58
IO3_SPARE  (via drill 0.3 pad 0.6)
  Top 0.2: v15.8,46.4 19,46.4 19.2,46.6 21.4,46.6 21.6,46.4 v22,46 | 53.4,28.2 53,28.6 52.8,28.8 52.6,29 52.4,29.2 52,29.6 51.8,29.8 51.6,30 51.4,30.2 51,30.6 50.8,30.8 50.6,31 50.4,31.2 50,31.6 49.8,31.8 49.6,32 49.4,32.2 49.2,32.4 49,32.6 48.8,32.8 48.6,33 v48.4,33.2 | v45.4,40.4 45,40.4 v44.2,41.2
  Top 0.25: U3.15 12.02,41.15
  Bottom 0.2: v12.4,45.6 15,45.6 15.2,45.8 15.4,46 15.6,46.2 v15.8,46.4 | v22,46 22.2,45.8 22.4,45.6 22.6,45.4 23,45 23.2,44.8 33.2,44.8 33.4,44.6 33.6,44.4 33.8,44.2 34,44 v34.2,43.8 | v48.4,33.2 48.2,33.4 48,33.6 47.8,33.8 47.6,34 47.4,34.2 47.2,34.4 47,34.6 46.8,34.8 46.6,35 46.4,35.2 46.2,35.4 46,35.6 46,37.2 45.6,37.6 45.4,37.8 v45.4,40.4 | v44.2,41.2 39.4,41.2 39.2,41.4 39,41.6 38.8,41.8 38.6,42 38.4,42.2 38.2,42.4 v35.8,42.4
LC_A_N  (via drill 0.3 pad 0.6)
  Top 0.2: 40.4,16 v40.4,15.8
  Bottom 0.2: v40.4,15.8 40.4,7.8 40.6,7.6 40.6,3.6
LC_A_P  (via drill 0.3 pad 0.6)
  Top 0.2: U8.8 40.3,15.3 42.3,11.8 | 42,11.6 v42,8.6 | v41,5.2 40.8,5 40.6,4.8 40.4,4.6 40,4.2 39.8,4 39.6,3.8 39.4,3.6
  Bottom 0.2: v42,8.6 42,6.2 41.8,6 41.6,5.8 41.4,5.6 v41,5.2
LDO_EN  (via drill 0.3 pad 0.6)
  Top 0.2: v12,16.2 8,16.2 | 8,16.2 7.8,16 7.4,15.6 7.2,15.4 7,15.2 6.8,15 6.4,14.6 6.2,14.4 6,14.2 5.8,14 5.4,13.6 5.2,13.4 5,13.2 4.8,13 4.4,12.6 4.2,12.4 4,12.2 3.8,12 3.6,11.8 3.4,11.6 3.2,11.4 3,11.2 | 7.2,22.8 7,22.6 6.8,22.6 6.8,19.6 7,19.4 7.2,19.2 7.4,19 7.6,18.8 7.6,16.6 7.8,16.4 8,16.2
  Bottom 0.2: v12,17.6 v12,16.2
LED_ALERT  (via drill 0.3 pad 0.6)
  Top 0.2: 44,57.2 42.8,57.2 42.6,57.4 41.6,57.4 41.4,57.2 41.2,57 41,56.8 40.8,56.6 40.6,56.4 40.4,56.2 v40.4,53.4 | v40.2,52.6 38.4,52.6 38.2,52.4 38,52.2 37.8,52 37.6,51.8 37,51.2 36.8,51 36.6,50.8 36.4,50.8 36.2,50.6 34.2,50.6 34,50.4 v33.8,50.4 | v32.4,50.4 v28.8,50.4 | v23.6,50.8 23.2,50.8 23,50.6 v22.8,50.4 | v17,48.8 16.8,48.6 16.6,48.4 16.4,48.2 16.2,48 16,47.8 15.8,47.6 14.2,47.6 v14,47.4 | v13.2,46.8 13.2,45.6
  Top 0.25: U3.16 13.29,39.45
  Bottom 0.2: v40.4,53.4 40.2,53.2 v40.2,52.6 | v33.8,50.4 v32.4,50.4 | v28.8,50.4 27.4,50.4 27.2,50.6 24,50.6 23.8,50.8 v23.6,50.8 | v22.8,50.4 18.6,50.4 18.4,50.2 18.2,50 18,49.8 17.8,49.6 17.6,49.4 17.4,49.2 17.2,49 v17,48.8 | v14,47.4 13.6,47 13.2,47 v13.2,46.8
LED_ALERT_A
  Top 0.2: 45.8,55.8 45.8,54.8
LED_CHRG_A  (via drill 0.3 pad 0.6)
  Top 0.2: 21.8,22.4 v21.8,21.6 | v22.4,19.8 17,19.8
  Bottom 0.2: v21.8,21.6 21.8,20.6 22,20.4 22.2,20.2 22.4,20 v22.4,19.8
LED_CHRG_K  (via drill 0.3 pad 0.6)
  Top 0.2: v19.8,22 19.8,22.4
  Top 0.25: U1.7 24.6,15.63
  Bottom 0.2: v22,16 22,17.8 21.6,18.2 21.4,18.4 21.2,18.6 21,18.8 20.8,19 20.6,19.2 20.2,19.6 20,19.8 19.8,20 v19.8,22
LED_STATUS  (via drill 0.3 pad 0.6)
  Top 0.2: 26.4,45.6 26.6,45.8 v26.6,46 | v30.8,49 31.8,49 32,49.2 32.6,49.8 32.8,50 33,50.2 33.6,50.8 33.8,51 34,51.2 34.6,51.8 34.6,52.2 34.8,52.4 34.8,52.6 35,52.8 35.2,53 35.4,53.2 35.6,53.4 35.8,53.6 36,53.8 36.2,54 36.4,54.2 36.6,54.4 36.8,54.6 37,54.8 37.2,55 37.4,55.2 37.6,55.4 37.8,55.6 38,55.8 38.2,56 38.4,56.2 38.6,56.4 38.8,56.6 39,56.8 39.2,57 39.4,57.2 39.6,57.4 39.8,57.6 40,57.8 40.2,58 40.4,58.2 40.6,58.4 40.8,58.6 41,58.8 41,59.6 41.2,59.8 41.2,60 41.4,60.2 41.6,60.2 41.8,60.4 v43,60.4
  Top 0.25: U3.26 25.98,42.85
  Bottom 0.2: v26.6,46 27.6,46 28,46.4 28.2,46.6 28.4,46.8 28.6,47 29,47.4 29.2,47.6 29.4,47.8 29.6,48 30,48.4 30.2,48.6 30.4,48.8 30.6,48.8 v30.8,49 | v43,60.4 43.6,60.4 43.8,60.6 v44,60.8
LED_STATUS_A  (via drill 0.3 pad 0.6)
  Top 0.2: 45.8,59.6 v45.8,60
  Bottom 0.2: v45.8,60 v45.8,60.8
LED_STDBY_A  (via drill 0.3 pad 0.6)
  Top 0.2: 20.8,24.8 20.6,24.6 20.6,24.4 18.4,24.4 18.2,24.6 17.8,25 v16.8,25
  Bottom 0.2: v16.8,25 v16.8,24.2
